(* Logix 5000 Rung export; software revision 16.04 *)

MODULES
   Local : vendor None type None code None
   MVI69E_AFC : vendor None type None code None
END_MODULES

TYPE AFCESiteAlarms :   // Indicates if a meter has any alarms
STRUCT
   Meter1 : BOOL;   // Meter in alarm
   Meter2 : BOOL;   // Meter in alarm
   Meter3 : BOOL;   // Meter in alarm
   Meter4 : BOOL;   // Meter in alarm
   Meter5 : BOOL;   // Meter in alarm
   Meter6 : BOOL;   // Meter in alarm
   Meter7 : BOOL;   // Meter in alarm
   Meter8 : BOOL;   // Meter in alarm
   Meter9 : BOOL;   // Meter in alarm
   Meter10 : BOOL;   // Meter in alarm
   Meter11 : BOOL;   // Meter in alarm
   Meter12 : BOOL;   // Meter in alarm
   Meter13 : BOOL;   // Meter in alarm
   Meter14 : BOOL;   // Meter in alarm
   Meter15 : BOOL;   // Meter in alarm
   Meter16 : BOOL;   // Meter in alarm
END_STRUCT
END_TYPE

TYPE AFCEFlag :   // Flags contains status information updated by ladder and also trigger bits for clock update
STRUCT
   AFCStopped : BOOL;   // Indicates that the module has sent a new input block to be processed by ladder - UPDATED BY LADDER
   AFCInputSequenceNum : INT;   // Meter number (0 -15) associated to blocks 1-16. Used to update "Profile" (meter type and product group.) UPDATED BY LADDER
END_STRUCT
END_TYPE

TYPE AFCEUtilBlockNonInterrupt :
STRUCT
   Now : BOOL;
   ModbusMasterCommand : BOOL;
   ModbusMasterResponse : BOOL;
   Archive : DINT;
   Prover : BOOL;
   PassThru : BOOL;
   Calibration : BOOL;
END_STRUCT
END_TYPE

TYPE AFCEProveConfigEnable :   // Prove controls at enable
STRUCT
   MeterNumber : INT;   // Meter number requested (1-16)
   AutoAcceptProve : BOOL;   // Auto-accept the prove
   AutoContinueProve : BOOL;   // Auto-continue the prove
END_STRUCT
END_TYPE

TYPE AFCEModbusGateway :   // Modbus Gateway
STRUCT
   Command : AFCEModbusGatewayCommand[10];   // Modbus gateway commands - contains setup and modbus data
END_STRUCT
END_TYPE

TYPE AFCEModbusMasterDataType :   // Modbus master data type
STRUCT
   Bit : BOOL;   // bit type
   Word : BOOL;   // word type (16-bit)
   Long : BOOL;   // long integer (32-bit)
   LongRemote : BOOL;   // long integer (32-bit)
END_STRUCT
END_TYPE

TYPE AFCEUtil :   // Used for internal ladder logic usage. These values must not be changed by user application.
STRUCT
   Flags : AFCEFlag;   // Wallclock update commands
   CycleCounter : INT;   // Reflects current block ID calculated by ladder to be sent to the module
   Buffer : AFCEUtilBuffer;
   Block : AFCEUtilBlock;
END_STRUCT
END_TYPE

TYPE AFCEWallclock :
STRUCT
   GetAFCTime : BOOL;   // Get current AFC Time
   SetAFCTimeFromPLCTime : BOOL;   // Set AFC time from PLC time. Updates current AFC time
   EnableLocalDateTime : BOOL;   // Enable Local Date Time.
   AFCTime : AFCETime;   // Coordinated Universal Time. Updated by either getting or setting AFC time.
END_STRUCT
END_TYPE

TYPE AFCEProvePhaseBitmap :   // AFC prove phase bitmap
STRUCT
   NotSelected : BOOL;   // Not selected
   Active : BOOL;   // Active, not counting
   CountingPast1stSwitch : BOOL;   // Counting past 1st switch for Udir and forward leg for Bdir)
   Past2ndSwitchFwdLeg : BOOL;   // Past 2nd switch forward leg (bidirectional only)
   Past1stSwithRetLeg : BOOL;   // Past 1st switch return leg (bidirectional only)
   RunComplete : BOOL;   // Run complete. past 2nd switch.
END_STRUCT
END_TYPE

TYPE AFCEProveInputConfig :   // Prove input block results - prover configuration
STRUCT
   Type : INT;   // Prover type
   Options : INT;   // Prover options
   RunsPerProveTotal : INT;   // Total runs per prove
   RunsPerProveSelected : INT;   // Selected runs per prove
   MaxRunsBeforeAbort : INT;   // Max total runs before abort
   ShortPassesPerRun : INT;   // Short passes per run if bidir = 2 , else 0
END_STRUCT
END_TYPE

TYPE AFCEModbusGatewayCommand :   // Modbus Gateway Command
STRUCT
   Config : AFCEModbusGatewayConfig;   // Config data to be entered by the user.
   Trigger : BOOL;   // Trigger the Command, when cleared module has responded.
   Data : INT[200];   // Contains modbus data written to the module (write commands)
END_STRUCT
END_TYPE

TYPE AFCEProveConfigAccept :   // Prove controls at accept. If auto-accept is selected must be available at enable
STRUCT
   RequestedInterpolationPoint : INT;   // Requested interpolation point (0 nearest)
   ApplyMFChangeAllStreams : BOOL;   // Apply change in meter factor to all streams
   ApplyMFChangeCurve : BOOL;   // Apply change in meter factor to all curve points
   ApplyNewMF : BOOL;   // CApply new meter factor
END_STRUCT
END_TYPE

TYPE AFCEModbusMasterCommand :   // Modbus Master Command
STRUCT
   Config : AFCEModbusMasterConfig;   // Modbus Master Configuration
   ErrorCode : INT;   // Error Code associated to Modbus Master Command
   Pending : BOOL;   // Pending Modbus Master Command - waiting for Modbus Response
   ReturnedTransactionID : DINT;   // Changes to Config.TransactionID value when response has returned.
   Data : INT[100];   // Read or Write Data
END_STRUCT
END_TYPE

TYPE AFCEProveSequencing :   // AFC prove sequencing tag for phase selection and ball positioning
STRUCT
   Phase : AFCEProvePhaseBitmap;   // AFC phase sequencing
   BallPositionReady : BOOL;   // Ball position: Ready (Udir & Bdir only; fwd leg Bdir)
   BallPositionSealed : BOOL;   // Ball position: Sealed (Udir & Bdir only; fwd leg Bdir)
   BallPositionReadyBwdLeg : BOOL;   // Ball position: Ready bwd leg (Bdir only)
   BallPositionSealedBwdLeg : BOOL;   // Ball position: Sealed bwd leg (Bdir only)
END_STRUCT
END_TYPE

TYPE AFCEUtilBlockInterrupt :
STRUCT
   Now : BOOL;
   ModbusGateway : DINT;
   EnableDisable : BOOL;
   Analysis : DINT;
END_STRUCT
END_TYPE

TYPE AFCEUtilBlock :
STRUCT
   ProcessInput : INT;
   InterruptPending : AFCEUtilBlockInterrupt;
   InterruptComplete : AFCEUtilBlockInterrupt;
   NonInterruptPending : AFCEUtilBlockNonInterrupt;
   NonInterruptComplete : AFCEUtilBlockNonInterrupt;
END_STRUCT
END_TYPE

TYPE AFCEModbusGatewayConfig :   // Modbus Ggateway Configuration
STRUCT
   Enable : BOOL;   // Set to 1 to enable modbus gateway command (0=disable)
   StartRegister : DINT;   // Start modbus address
   RegisterCount : INT;   // Word count (200 max)
   FunctionType : BOOL;   // 0 = read command, 1 = write command
   RegisterType : BOOL;   // 0 = holding register, 1 = input register
   SlaveType : BOOL;   // 0 = primary slave, 1 = virtual slave
END_STRUCT
END_TYPE

TYPE AFCEModbusPassThru :   // AFC Modbus Pass-thru
STRUCT
   Enable : BOOL;   // Set to 1 to enable pass-thru functionality (requires AFC Manager setting)
   MessagePresent : BOOL;   // Message present in the response block
   GetMessage : BOOL;   // Get the pass-thru message. When the bit is cleared the message has been transferred to the PLC.
   FunctionBitWrite : BOOL;   // Function bit write
   OverflowError : BOOL;   // Overflow error flag
   ModbusAddress : INT;   // Destination modbus address
   RegisterCount : INT;   // Number of elements associated to command
   ReadDataWord : INT[125];   // Contains received data for word commands
   ReadDataBit : AFCEModbusPassThruBitData;   // Contains received data for bit commands
END_STRUCT
END_TYPE

TYPE AFCEUtilBuffer :   // Buffer
STRUCT
   Input : INT[248];   // Input buffer contains the complete block to be copied from the module
   Output : INT[247];   // Output buffer contains data the complete block to be copied to the module
   Process : INT[180];
   ArchiveDay : INT[98];
   ArchiveHour : INT[98];
   Prove : INT[26];
   Analysis : INT[198];
   MeterEnableDisable : INT[4];
   StreamEnable : INT[36];
   StreamDisable : INT[36];
   StreamSelect : INT[24];
   MeterSignals : INT[24];
   Calibration : INT[36];
END_STRUCT
END_TYPE

TYPE AFCEProveStatus :   // Status of the prove (returned from the module to the processor)
STRUCT
   ProveAccepted : BOOL;   // Prove was accepted
   MeterFactorApplied : BOOL;   // Meter factor was applied
   MFAppliedToCurve : BOOL;   // Meter factor was applied to all points in the curve
   MFAppliedToStreams : BOOL;   // Meter factor was applied to all streams
   ProveRejectedByCommand : BOOL;   // Prove was rejected by command
   ProveRejectedNoRuns : BOOL;   // Prove was rejected - empty prove (no runs)
   ProveRejectedDivideBy0 : BOOL;   // Prove was rejected - divide by 0
   ProveEnabled : BOOL;   // Prove is enabled
   ProvingRunInProgress : BOOL;   // Proving run is in progress
   ProveRejectedAbort : BOOL;   // Prove rejected: abort
   ProvePaused : BOOL;   // Prove is paused
   RunCancelled : BOOL;   // Run Is cancelled
   RunTimedOut : BOOL;   // Run timed out
END_STRUCT
END_TYPE

TYPE AFCEProveConfig :   // Controls (configuration settings) associated to the prover
STRUCT
   Enable : AFCEProveConfigEnable;   // Controls at enable
   Accept : AFCEProveConfigAccept;   // Controls at accept
END_STRUCT
END_TYPE

TYPE AFCESiteStatus :   // Site status bits - contains general information about the module - not meter specific
STRUCT
   AFCActive : BOOL;   // AFC active
   ChecksumAlarms : BOOL;   // Checkum alarm active
   Reserved2 : BOOL;
   Reserved3 : BOOL;
   PLCHalted : BOOL;   // PLC in program mode or missing
   CfgChanged : BOOL;   // Configuration changed
   Powerup : BOOL;   // Module powered up
   ColdStart : BOOL;   // Module performed cold start (BBRAM initialized)
   ModbusMasterPending : BOOL;   // Modbus Master Poll Pending
   ModbusMasterComplete : BOOL;   // Modbus Master Poll Complete
   ModbusPassThruPending : BOOL;   // Modbus Pass-thru Input Pending
   CalibrationRequest : BOOL;   // Calibration request from module
   ProverEnabled : BOOL;   // Prover Enabled
   Reserved13 : BOOL;
   Reserved14 : BOOL;
   Reserved15 : BOOL;
END_STRUCT
END_TYPE

TYPE AFCEModbusMaster :   // Modbus Master. Port 3 must be configured as modbus master through AFC Manager to use this feature.
STRUCT
   Enable : BOOL;   // Enable the modbus master funcionality
   CommandIndex : INT;   // Selects which command index will be executed
   Command : AFCEModbusMasterCommand[10];   // Each command contains a specific modbus request to be sent out of the port
END_STRUCT
END_TYPE

TYPE AFCEProveProcess :   // Prove process output from processor to the module
STRUCT
   Sequencing : AFCEProveSequencing;   // Prover sequencing
   Temperature : REAL;   // Temperature for Single Probe provers. And Inlet Temperature for Dual Probe Provers.
   OutletTemperature : REAL;   // Outlet Temperature for Provers with Dual Probes.
   SwitchBarTemperature : REAL;   // Switch bar temperature
   Pressure : REAL;   // Pressure for Single Probe provers. And Inlet Pressure for Dual Probe Provers.
   OutletPressure : REAL;   // Outlet Pressure for Provers with Dual Probes.
   ProverDensity : REAL;   // Prover density
END_STRUCT
END_TYPE

TYPE AFCETime :   // AFC time format used for wallclock update.
STRUCT
   Year : DINT;   // Year
   Month : DINT;   // Month
   Day : DINT;   // Day
   Hour : DINT;   // Hour
   Minute : DINT;   // Minute
   second : DINT;   // Seconds
END_STRUCT
END_TYPE

TYPE AFCEModbusMasterSwap :   // Modbus master swap words/ swap bytes
STRUCT
   SwapWords : BOOL;   // Swap words
   SwapBytes : BOOL;   // Swap bytes
END_STRUCT
END_TYPE

TYPE AFCEProvePulseCount :   // Values to be supplied at the end of the pass/run
STRUCT
   Meter : DINT;   // Meter pulse count
   MasterMeter : DINT;   // Master meter pulse count
END_STRUCT
END_TYPE

TYPE AFCEModbusPassThruBitData :   // AFC Modbus Pass-thru Bit Data
STRUCT
   Data : BOOL[2016];   // Contains received data for bit commands
END_STRUCT
END_TYPE

TYPE AFCEModbusMasterConfig :   // Modbus master command settings
STRUCT
   Enable : BOOL;   // Set to 1 to enable command (0=disable)
   FunctionType : BOOL;   // Set to 1 to select write command (0=read command)
   RegisterBank : BOOL;   // Set to 1 to select input register (0=holding register)
   DataType : AFCEModbusMasterDataType;   // Select data type format
   SwapOption : AFCEModbusMasterSwap;   // Select byte and word swap (1 = swap, 0 = no swap)
   TypeSwap : INT;   // This value is calculated by ladder logic and must not be modified by user
   SlaveAddress : INT;   // Modbus slave address of remote device
   ModbusAddress : INT;   // Modbus data address on remote slave
   ElementCount : INT;   // Number of data elements (125 words)
   TransactionID : INT;   // Transaction ID. This value is returned to the ReturnedTransaction ID when the response has been received.
END_STRUCT
END_TYPE

TYPE AFCEModuleDef :   // Main user defined data type
STRUCT
   ModbusGateway : AFCEModbusGateway;   // Reads and write data between processor and module modbus table
   ModbusMaster : AFCEModbusMaster;   // Setup modbus master commands to be sent to remote slaves (through Port 3)
   ModbusPassThru : AFCEModbusPassThru;   // Modbus pass-thru data
   SiteStatus : AFCESiteStatus;   // Site status
   MeterAlarms : AFCESiteAlarms;   // Meter Alarms
   Prove : AFCEProve;   // Prover
   Wallclock : AFCEWallclock;   // Set clock and get clock information
   Firmware : AFCEFirmwareVersion;   // Firmware information
   Util : AFCEUtil;   // Used by ladder logic
END_STRUCT
END_TYPE

TYPE AFCEProveSignals :   // Contains the proving signals that will trigger specific tasks from the module
STRUCT
   EnableProve : BOOL;   // Enables the prove
   AcceptProve : BOOL;   // Accepts the prove
   RejectProve : BOOL;   // Reject the prove
   RunStart : BOOL;   // Starts the run
   RunComplete : BOOL;   // Flags that the run is complete
   RunCancel : BOOL;   // Cancels the run
   RunDelete : BOOL;   // Deletes the run
   PassComplete : BOOL;   // Flag that the pass is complete
   PauseProve : BOOL;   // Pauses the Proving Process
   AbortProve : BOOL;   // Aborts the prove
END_STRUCT
END_TYPE

TYPE AFCEFirmwareVersion :
STRUCT
   Major : SINT;   // Major Version number
   Minor : SINT;   // Minor Version number
   Revision : INT;   // Revision
END_STRUCT
END_TYPE

TYPE AFCEProveRunResults :   // Run results of the prove. Copied from the module to the pocessor
STRUCT
   CountAttempted : INT;   // Run count attempted
   CountCompleted : INT;   // Run count completed
   CountSelected : INT;   // Run count selected
   RunsSelected : INT;   // Bit Mapped Runs selected for calculations from completed runs
   NewMeterFactor : REAL;   // New meter factor
   ChangeInMeterFactor : REAL;   // Change in meter factor
END_STRUCT
END_TYPE

TYPE AFCEProve :   // Prove
STRUCT
   Process : AFCEProveProcess;   // Process Variables
   Signals : AFCEProveSignals;   // AFC Prove Signals (triggers the proving update)
   Config : AFCEProveConfig;   // AFC Prove Control (configuration settings)
   PulseCounts : AFCEProvePulseCount;   // Pulse counts to be updated at the end of the run/pass
   ConfigInput : AFCEProveInputConfig;   // AFC prover input configuration
   Status : AFCEProveStatus;   // AFC prover status
   ErrorCode : INT;   // Prove error code
   ProveControlsEcho : INT;   // AFC module Echos the state of the Prove Controls
   RequestedMeterEcho : INT;   // AFC module Echos the Meter number requested
   RequestedCurvePointEcho : INT;   // AFC module Echos the requested Curve Point
   RunResults : AFCEProveRunResults;   // Prove and run results
   ProveEnabled : BOOL;   // ON if prove is enabled. This flag is coped from inputbuffer[247]
END_STRUCT
END_TYPE

ADD_ON_INSTRUCTION AOI69EAFC   (* revision 1.5, vendor ProSoft Technology Inc., ExecutePrescan *)
// Add-On instruction for the MVI69E-AFC.
// Module Interface.
// Revision note:
// Made changes to the ModbusGatewayConfig UDT StartRegister Tag Data Type from INT to DINT.
// Help:
// Compatible with version 4.04 of MVI69E-AFC firmware or higher.
// v1.3: Option to choose LocalDateTime.
// v1.4: Changed Prescan FLL instruction length from 240 words to 180 for proccess inputs. This stopped mismatch issue
// v1.4: Changed COP instruction length from 240 words to 180 on rung 19 for procces inputs to output block. Modified ProfileBlockID INT to DINT.
// v1.5: Made changes to the ModbusGatewayConfig UDT StartRegister Tag Data Type from INT to DINT.
VAR_IN_OUT
   ConnectionInput : INT[248]; {required}
   ConnectionOutput : INT[247]; {required}
   AFC : AFCEModuleDef; {required}
        .UTIL.BUFFER.PROVE[12]   // Main user defined data type Buffer
END_VAR
VAR
   WallclockCurrentPLCTime : DINT[7];
   UTCTimeDelta : DINT;
   TimeZoneString : STRING;
   StoppedTimer : TIMER;
   ProverSignals : DINT;
   ProverPhase : DINT;
   ProverControls : DINT;
   ProveEnabled : BOOL;
   ProfileBlockID : DINT;
   ModbusMasterOutput : INT;
   CycleCounterPreviousStopped : INT;
   Offset1 : DINT;
   NotStoppedTimer : TIMER;
   ModbusPassThruOverflowError : BOOL;
   ModbusPassThruOutput : DINT;
   ModbusPassThruMessagePresent : BOOL;
   ModbusPassThruFunctionBitWrite : BOOL;
   ModbusMasterTransactionNumber : DINT;
   ModbusMasterReadWrite : BOOL;   // 0=Read 1=Write
   ModbusMasterPending : BOOL;
   ModbusMasterLongCount : DINT;
   ModbusGatewayReadWrite : BOOL;   // 0=Read, 1=Write
   ModbusGatewayOutput : DINT;
   ModbusGatewayIndexBitPosition : DINT;
   ModbusGatewayIndex : DINT;
   MJFAULTS : DINT[12];
   LocalHourChange : DINT;
   LatchStopped : BOOL;
   ForceReset : BOOL;
   AvoidBufferOverflowFault : DINT;   // Need this to prevent Overflow Minor Fault
   AFCTime : AFCETime;
END_VAR

ROUTINE Logic   (* ladder *)
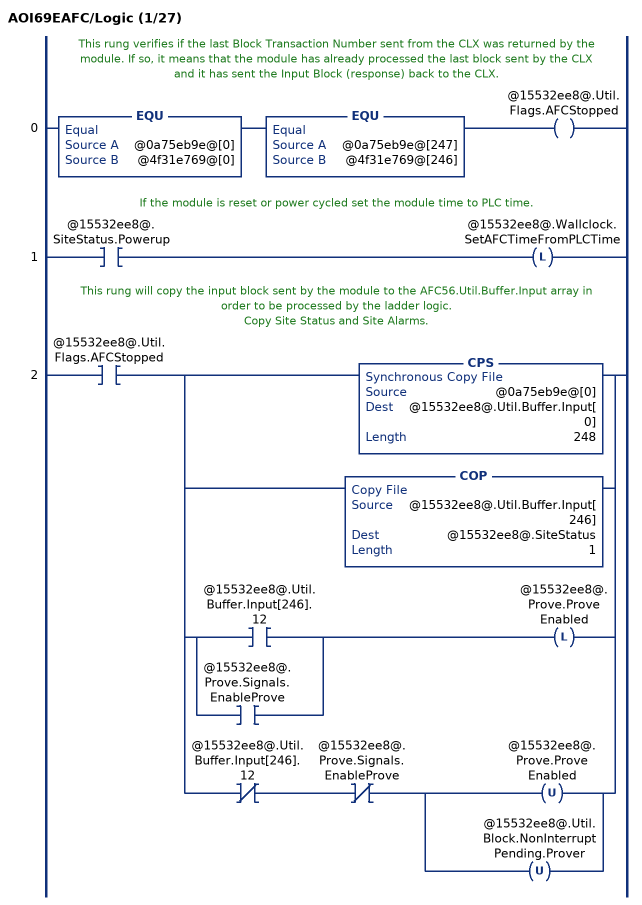
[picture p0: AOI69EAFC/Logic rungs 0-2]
   // This rung verifies if the last Block Transaction Number sent from the CLX was returned by the module. If so, it means that the module has already processed the last block sent by the CLX and it has sent the Input Block (response) back to the CLX.
   0: EQU(@0a75eb9e@[0],@4f31e769@[0])EQU(@0a75eb9e@[247],@4f31e769@[246])OTE(@15532ee8@.Util.Flags.AFCStopped);
   // If the module is reset or power cycled set the module time to PLC time.
   1: XIC(@15532ee8@.SiteStatus.Powerup)OTL(@15532ee8@.Wallclock.SetAFCTimeFromPLCTime);
   // This rung will copy the input block sent by the module to the AFC56.Util.Buffer.Input array in order to be processed by the ladder logic.
   // Copy Site Status and Site Alarms.
   2: XIC(@15532ee8@.Util.Flags.AFCStopped)[CPS(@0a75eb9e@[0],@15532ee8@.Util.Buffer.Input[0],248) ,COP(@15532ee8@.Util.Buffer.Input[246],@15532ee8@.SiteStatus,1) ,[XIC(@15532ee8@.Util.Buffer.Input[246].12) ,XIC(@15532ee8@.Prove.Signals.EnableProve) ] OTL(@15532ee8@.Prove.ProveEnabled) ,XIO(@15532ee8@.Util.Buffer.Input[246].12) XIO(@15532ee8@.Prove.Signals.EnableProve) [OTU(@15532ee8@.Prove.ProveEnabled) ,OTU(@15532ee8@.Util.Block.NonInterruptPending.Prover) ] ];
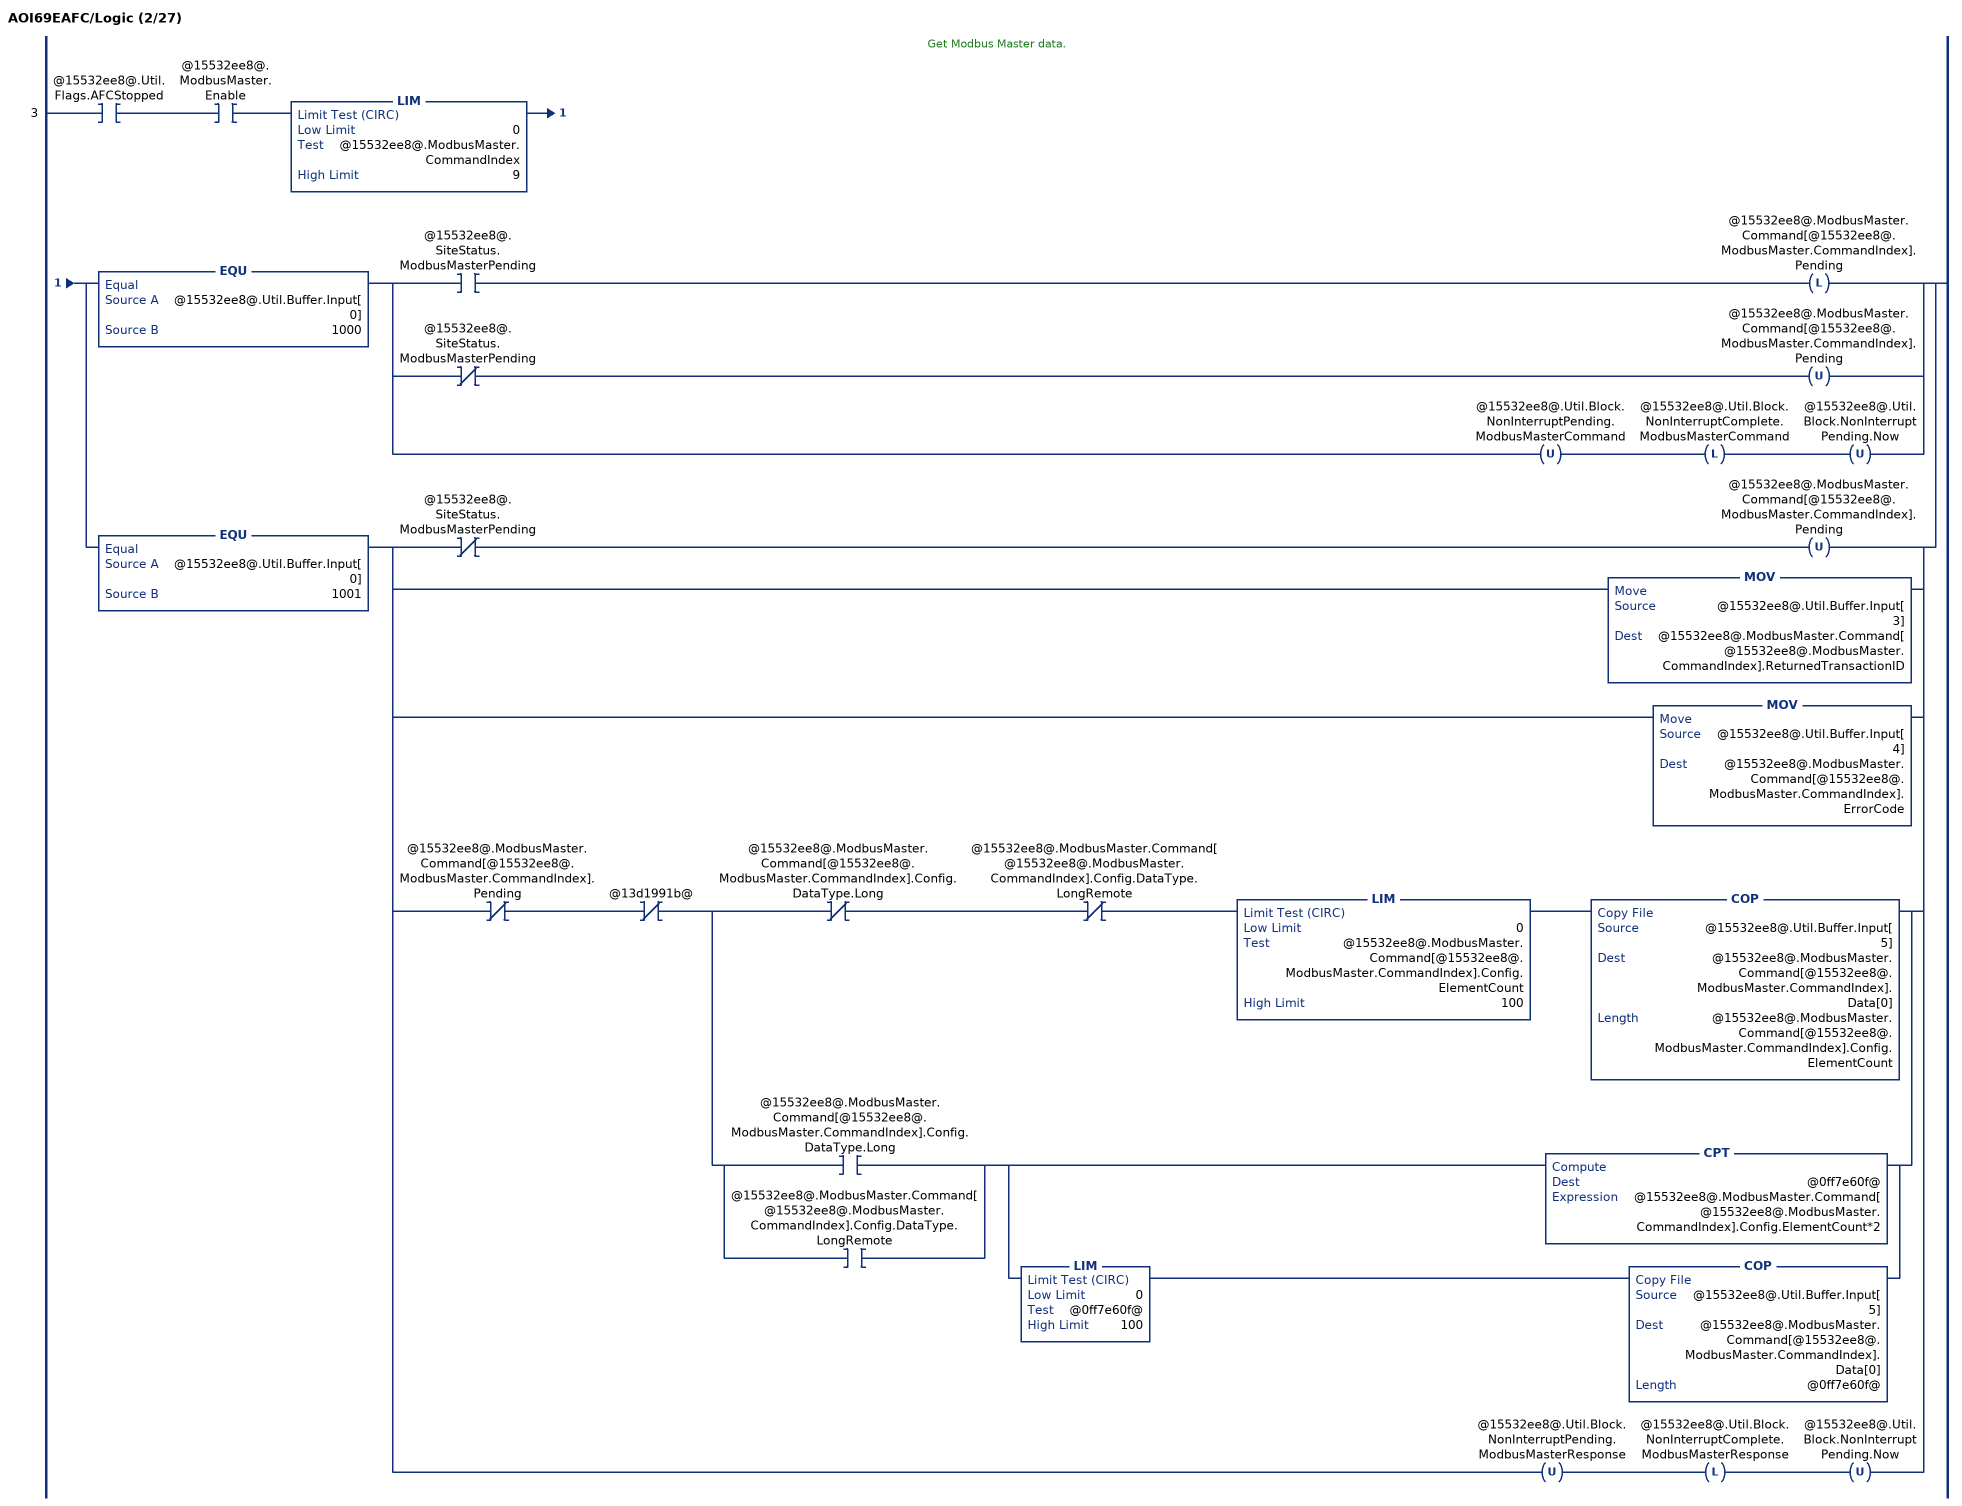
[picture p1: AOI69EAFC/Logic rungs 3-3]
   // Get Modbus Master data.
   3: XIC(@15532ee8@.Util.Flags.AFCStopped)XIC(@15532ee8@.ModbusMaster.Enable)LIM(0,@15532ee8@.ModbusMaster.CommandIndex,9)[EQU(@15532ee8@.Util.Buffer.Input[0],1000) [XIC(@15532ee8@.SiteStatus.ModbusMasterPending) OTL(@15532ee8@.ModbusMaster.Command[@15532ee8@.ModbusMaster.CommandIndex].Pending) ,XIO(@15532ee8@.SiteStatus.ModbusMasterPending) OTU(@15532ee8@.ModbusMaster.Command[@15532ee8@.ModbusMaster.CommandIndex].Pending) ,OTU(@15532ee8@.Util.Block.NonInterruptPending.ModbusMasterCommand) OTL(@15532ee8@.Util.Block.NonInterruptComplete.ModbusMasterCommand) OTU(@15532ee8@.Util.Block.NonInterruptPending.Now) ] ,EQU(@15532ee8@.Util.Buffer.Input[0],1001) [XIO(@15532ee8@.SiteStatus.ModbusMasterPending) OTU(@15532ee8@.ModbusMaster.Command[@15532ee8@.ModbusMaster.CommandIndex].Pending) ,MOV(@15532ee8@.Util.Buffer.Input[3],@15532ee8@.ModbusMaster.Command[@15532ee8@.ModbusMaster.CommandIndex].ReturnedTransactionID) ,MOV(@15532ee8@.Util.Buffer.Input[4],@15532ee8@.ModbusMaster.Command[@15532ee8@.ModbusMaster.CommandIndex].ErrorCode) ,XIO(@15532ee8@.ModbusMaster.Command[@15532ee8@.ModbusMaster.CommandIndex].Pending) XIO(@13d1991b@) [XIO(@15532ee8@.ModbusMaster.Command[@15532ee8@.ModbusMaster.CommandIndex].Config.DataType.Long) XIO(@15532ee8@.ModbusMaster.Command[@15532ee8@.ModbusMaster.CommandIndex].Config.DataType.LongRemote) LIM(0,@15532ee8@.ModbusMaster.Command[@15532ee8@.ModbusMaster.CommandIndex].Config.ElementCount,100) COP(@15532ee8@.Util.Buffer.Input[5],@15532ee8@.ModbusMaster.Command[@15532ee8@.ModbusMaster.CommandIndex].Data[0],@15532ee8@.ModbusMaster.Command[@15532ee8@.ModbusMaster.CommandIndex].Config.ElementCount) ,[XIC(@15532ee8@.ModbusMaster.Command[@15532ee8@.ModbusMaster.CommandIndex].Config.DataType.Long) ,XIC(@15532ee8@.ModbusMaster.Command[@15532ee8@.ModbusMaster.CommandIndex].Config.DataType.LongRemote) ] [CPT(@0ff7e60f@,@15532ee8@.ModbusMaster.Command[@15532ee8@.ModbusMaster.CommandIndex].Config.ElementCount*2) ,LIM(0,@0ff7e60f@,100) COP(@15532ee8@.Util.Buffer.Input[5],@15532ee8@.ModbusMaster.Command[@15532ee8@.ModbusMaster.CommandIndex].Data[0],@0ff7e60f@) ] ] ,OTU(@15532ee8@.Util.Block.NonInterruptPending.ModbusMasterResponse) OTL(@15532ee8@.Util.Block.NonInterruptComplete.ModbusMasterResponse) OTU(@15532ee8@.Util.Block.NonInterruptPending.Now) ] ];
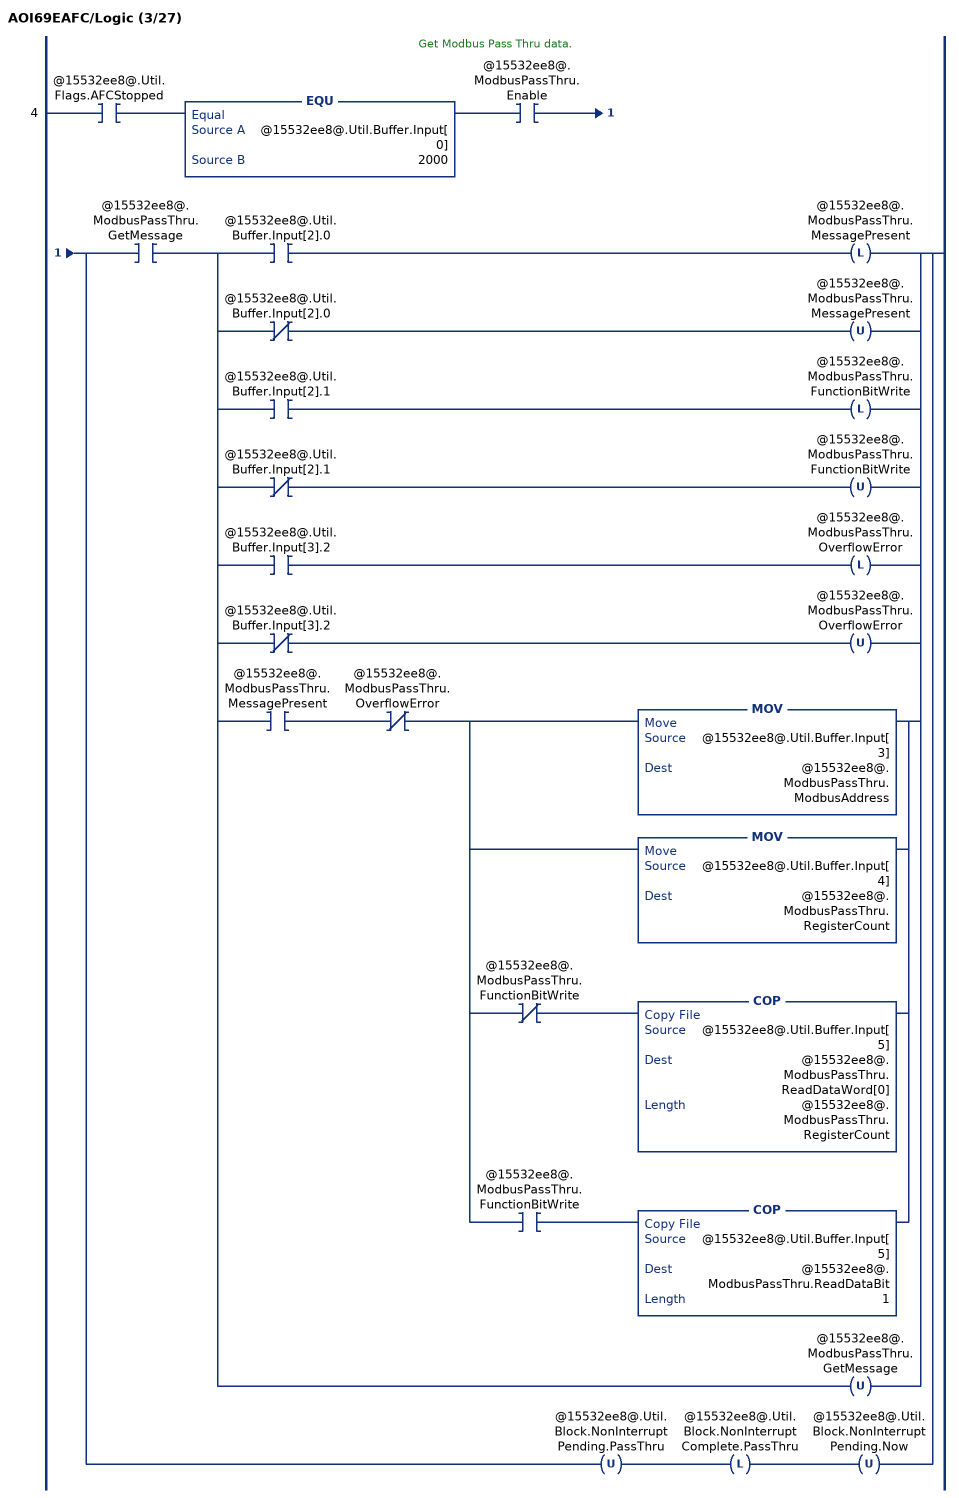
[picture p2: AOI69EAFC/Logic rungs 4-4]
   // Get Modbus Pass Thru data.
   4: XIC(@15532ee8@.Util.Flags.AFCStopped)EQU(@15532ee8@.Util.Buffer.Input[0],2000)XIC(@15532ee8@.ModbusPassThru.Enable)[XIC(@15532ee8@.ModbusPassThru.GetMessage) [[XIC(@15532ee8@.Util.Buffer.Input[2].0) OTL(@15532ee8@.ModbusPassThru.MessagePresent) ,XIO(@15532ee8@.Util.Buffer.Input[2].0) OTU(@15532ee8@.ModbusPassThru.MessagePresent) ,XIC(@15532ee8@.Util.Buffer.Input[2].1) OTL(@15532ee8@.ModbusPassThru.FunctionBitWrite) ,XIO(@15532ee8@.Util.Buffer.Input[2].1) OTU(@15532ee8@.ModbusPassThru.FunctionBitWrite) ,XIC(@15532ee8@.Util.Buffer.Input[3].2) OTL(@15532ee8@.ModbusPassThru.OverflowError) ,XIO(@15532ee8@.Util.Buffer.Input[3].2) OTU(@15532ee8@.ModbusPassThru.OverflowError) ] ,XIC(@15532ee8@.ModbusPassThru.MessagePresent) XIO(@15532ee8@.ModbusPassThru.OverflowError) [MOV(@15532ee8@.Util.Buffer.Input[3],@15532ee8@.ModbusPassThru.ModbusAddress) ,MOV(@15532ee8@.Util.Buffer.Input[4],@15532ee8@.ModbusPassThru.RegisterCount) ,XIO(@15532ee8@.ModbusPassThru.FunctionBitWrite) COP(@15532ee8@.Util.Buffer.Input[5],@15532ee8@.ModbusPassThru.ReadDataWord[0],@15532ee8@.ModbusPassThru.RegisterCount) ,XIC(@15532ee8@.ModbusPassThru.FunctionBitWrite) COP(@15532ee8@.Util.Buffer.Input[5],@15532ee8@.ModbusPassThru.ReadDataBit,1) ] ,OTU(@15532ee8@.ModbusPassThru.GetMessage) ] ,OTU(@15532ee8@.Util.Block.NonInterruptPending.PassThru) OTL(@15532ee8@.Util.Block.NonInterruptComplete.PassThru) OTU(@15532ee8@.Util.Block.NonInterruptPending.Now) ];
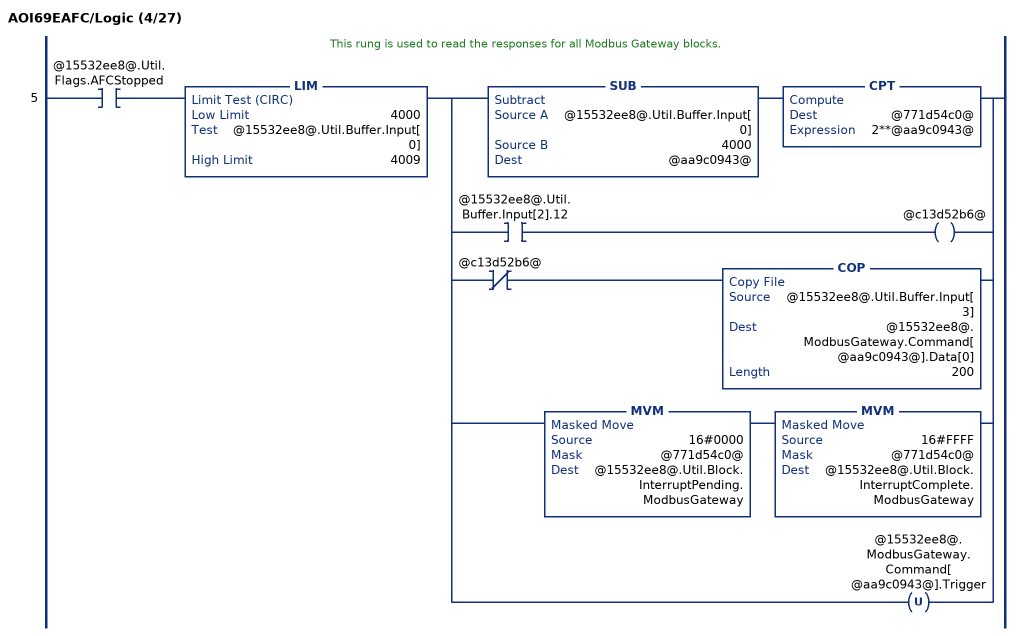
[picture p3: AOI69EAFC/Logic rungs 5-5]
   // This rung is used to read the responses for all Modbus Gateway blocks.
   5: XIC(@15532ee8@.Util.Flags.AFCStopped)LIM(4000,@15532ee8@.Util.Buffer.Input[0],4009)[SUB(@15532ee8@.Util.Buffer.Input[0],4000,@aa9c0943@) CPT(@771d54c0@,2**@aa9c0943@) ,XIC(@15532ee8@.Util.Buffer.Input[2].12) OTE(@c13d52b6@) ,XIO(@c13d52b6@) COP(@15532ee8@.Util.Buffer.Input[3],@15532ee8@.ModbusGateway.Command[@aa9c0943@].Data[0],200) ,MVM(16#0000,@771d54c0@,@15532ee8@.Util.Block.InterruptPending.ModbusGateway) MVM(16#FFFF,@771d54c0@,@15532ee8@.Util.Block.InterruptComplete.ModbusGateway) ,OTU(@15532ee8@.ModbusGateway.Command[@aa9c0943@].Trigger) ];
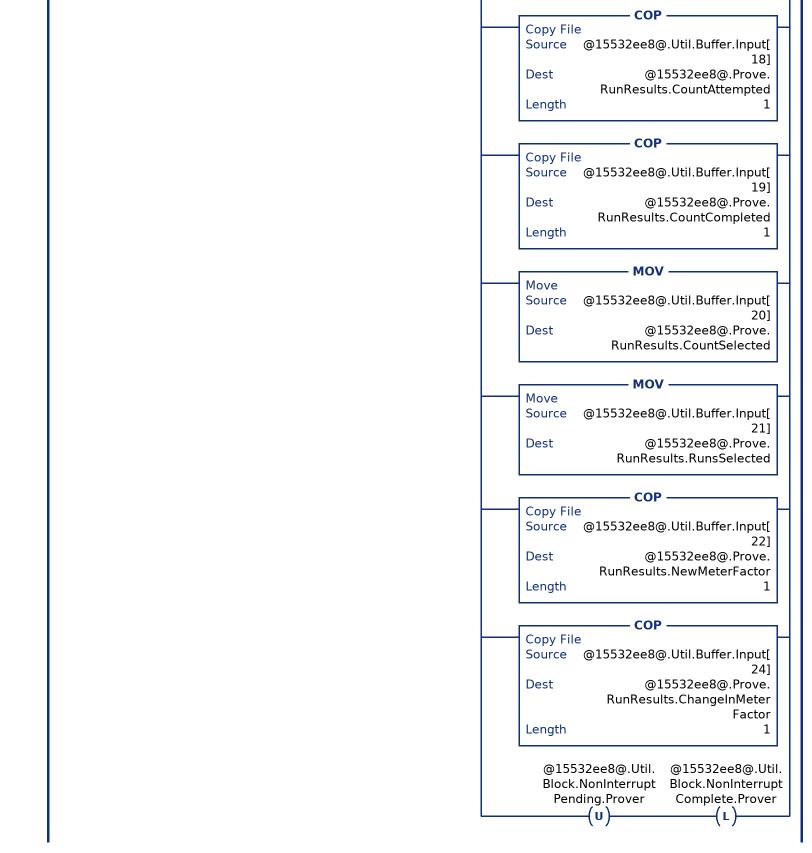
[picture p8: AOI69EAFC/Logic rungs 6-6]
   6: XIC(@15532ee8@.Util.Flags.AFCStopped)EQU(@15532ee8@.Util.Buffer.Input[0],5000)[XIC(@f8aaafbf@.1) OTU(@15532ee8@.Prove.Signals.EnableProve) ,XIC(@f8aaafbf@.2) OTU(@15532ee8@.Prove.Signals.AcceptProve) ,XIC(@f8aaafbf@.3) OTU(@15532ee8@.Prove.Signals.RejectProve) ,XIC(@f8aaafbf@.4) OTU(@15532ee8@.Prove.Signals.RunStart) ,XIC(@f8aaafbf@.5) OTU(@15532ee8@.Prove.Signals.RunComplete) ,XIC(@f8aaafbf@.6) OTU(@15532ee8@.Prove.Signals.RunCancel) ,XIC(@f8aaafbf@.7) OTU(@15532ee8@.Prove.Signals.RunDelete) ,XIC(@f8aaafbf@.9) OTU(@15532ee8@.Prove.Signals.PassComplete) ,XIC(@f8aaafbf@.12) OTU(@15532ee8@.Prove.Signals.PauseProve) ,XIC(@f8aaafbf@.14) OTU(@15532ee8@.Prove.Signals.AbortProve) ,MOV(@15532ee8@.Util.Buffer.Input[3],@15532ee8@.Prove.ConfigInput.Type) ,MOV(@15532ee8@.Util.Buffer.Input[4],@15532ee8@.Prove.ConfigInput.Options) ,MOV(@15532ee8@.Util.Buffer.Input[5],@15532ee8@.Prove.ConfigInput.RunsPerProveTotal) ,MOV(@15532ee8@.Util.Buffer.Input[6],@15532ee8@.Prove.ConfigInput.RunsPerProveSelected) ,MOV(@15532ee8@.Util.Buffer.Input[7],@15532ee8@.Prove.ConfigInput.MaxRunsBeforeAbort) ,MOV(@15532ee8@.Util.Buffer.Input[8],@15532ee8@.Prove.ConfigInput.ShortPassesPerRun) ,XIC(@15532ee8@.Util.Buffer.Input[12].0) OTL(@15532ee8@.Prove.Status.ProveAccepted) ,XIO(@15532ee8@.Util.Buffer.Input[12].0) OTU(@15532ee8@.Prove.Status.ProveAccepted) ,XIC(@15532ee8@.Util.Buffer.Input[12].1) OTL(@15532ee8@.Prove.Status.MeterFactorApplied) ,XIO(@15532ee8@.Util.Buffer.Input[12].1) OTU(@15532ee8@.Prove.Status.MeterFactorApplied) ,XIC(@15532ee8@.Util.Buffer.Input[12].2) OTL(@15532ee8@.Prove.Status.MFAppliedToCurve) ,XIO(@15532ee8@.Util.Buffer.Input[12].2) OTU(@15532ee8@.Prove.Status.MFAppliedToCurve) ,XIC(@15532ee8@.Util.Buffer.Input[12].3) OTL(@15532ee8@.Prove.Status.MFAppliedToStreams) ,XIO(@15532ee8@.Util.Buffer.Input[12].3) OTU(@15532ee8@.Prove.Status.MFAppliedToStreams) ,XIC(@15532ee8@.Util.Buffer.Input[12].4) OTL(@15532ee8@.Prove.Status.ProveRejectedByCommand) ,XIO(@15532ee8@.Util.Buffer.Input[12].4) OTU(@15532ee8@.Prove.Status.ProveRejectedByCommand) ,XIC(@15532ee8@.Util.Buffer.Input[12].5) OTL(@15532ee8@.Prove.Status.ProveRejectedNoRuns) ,XIO(@15532ee8@.Util.Buffer.Input[12].5) OTU(@15532ee8@.Prove.Status.ProveRejectedNoRuns) ,XIC(@15532ee8@.Util.Buffer.Input[12].6) OTL(@15532ee8@.Prove.Status.ProveRejectedDivideBy0) ,XIO(@15532ee8@.Util.Buffer.Input[12].6) OTU(@15532ee8@.Prove.Status.ProveRejectedDivideBy0) ,XIC(@15532ee8@.Util.Buffer.Input[12].8) OTL(@15532ee8@.Prove.Status.ProveEnabled) ,[XIO(@15532ee8@.Util.Buffer.Input[12].8) ,XIC(@f8aaafbf@.2) ,XIC(@f8aaafbf@.3) ,XIC(@f8aaafbf@.14) ] OTU(@15532ee8@.Prove.Status.ProveEnabled) ,XIC(@15532ee8@.Util.Buffer.Input[12].9) OTL(@15532ee8@.Prove.Status.ProvingRunInProgress) ,XIO(@15532ee8@.Util.Buffer.Input[12].9) OTU(@15532ee8@.Prove.Status.ProvingRunInProgress) ,XIC(@15532ee8@.Util.Buffer.Input[12].10) OTL(@15532ee8@.Prove.Status.ProvePaused) ,XIO(@15532ee8@.Util.Buffer.Input[12].10) OTU(@15532ee8@.Prove.Status.ProvePaused) ,XIC(@15532ee8@.Util.Buffer.Input[12].11) OTL(@15532ee8@.Prove.Status.RunCancelled) ,XIO(@15532ee8@.Util.Buffer.Input[12].11) OTU(@15532ee8@.Prove.Status.RunCancelled) ,XIC(@15532ee8@.Util.Buffer.Input[12].12) OTL(@15532ee8@.Prove.Status.RunTimedOut) ,XIO(@15532ee8@.Util.Buffer.Input[12].12) OTU(@15532ee8@.Prove.Status.RunTimedOut) ,XIC(@15532ee8@.Util.Buffer.Input[12].14) OTL(@15532ee8@.Prove.Status.ProveRejectedAbort) ,XIO(@15532ee8@.Util.Buffer.Input[12].14) OTU(@15532ee8@.Prove.Status.ProveRejectedAbort) ,MOV(@15532ee8@.Util.Buffer.Input[13],@15532ee8@.Prove.ErrorCode) ,MOV(@15532ee8@.Util.Buffer.Input[14],@15532ee8@.Prove.ProveControlsEcho) ,MOV(@15532ee8@.Util.Buffer.Input[15],@15532ee8@.Prove.RequestedMeterEcho) ,MOV(@15532ee8@.Util.Buffer.Input[17],@15532ee8@.Prove.RequestedCurvePointEcho) ,COP(@15532ee8@.Util.Buffer.Input[18],@15532ee8@.Prove.RunResults.CountAttempted,1) ,COP(@15532ee8@.Util.Buffer.Input[19],@15532ee8@.Prove.RunResults.CountCompleted,1) ,MOV(@15532ee8@.Util.Buffer.Input[20],@15532ee8@.Prove.RunResults.CountSelected) ,MOV(@15532ee8@.Util.Buffer.Input[21],@15532ee8@.Prove.RunResults.RunsSelected) ,COP(@15532ee8@.Util.Buffer.Input[22],@15532ee8@.Prove.RunResults.NewMeterFactor,1) ,COP(@15532ee8@.Util.Buffer.Input[24],@15532ee8@.Prove.RunResults.ChangeInMeterFactor,1) ,OTU(@15532ee8@.Util.Block.NonInterruptPending.Prover) OTL(@15532ee8@.Util.Block.NonInterruptComplete.Prover) ];
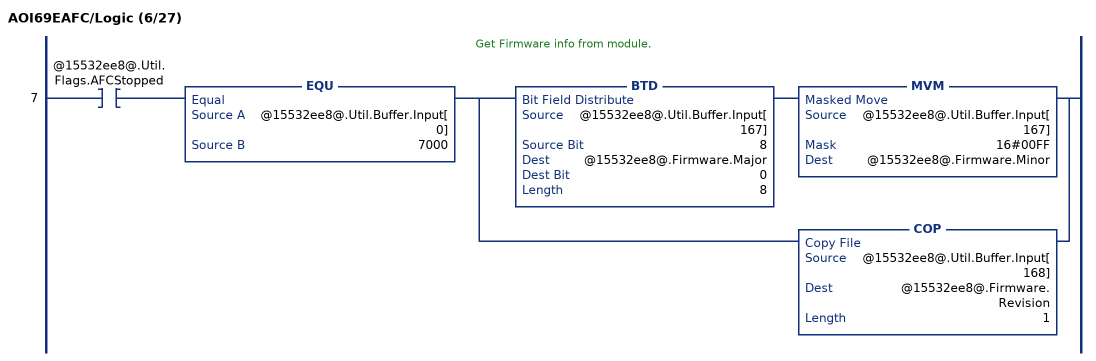
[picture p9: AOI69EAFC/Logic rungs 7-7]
   // Get Firmware info from module.
   7: XIC(@15532ee8@.Util.Flags.AFCStopped)EQU(@15532ee8@.Util.Buffer.Input[0],7000)[BTD(@15532ee8@.Util.Buffer.Input[167],8,@15532ee8@.Firmware.Major,0,8) MVM(@15532ee8@.Util.Buffer.Input[167],16#00FF,@15532ee8@.Firmware.Minor) ,COP(@15532ee8@.Util.Buffer.Input[168],@15532ee8@.Firmware.Revision,1) ];
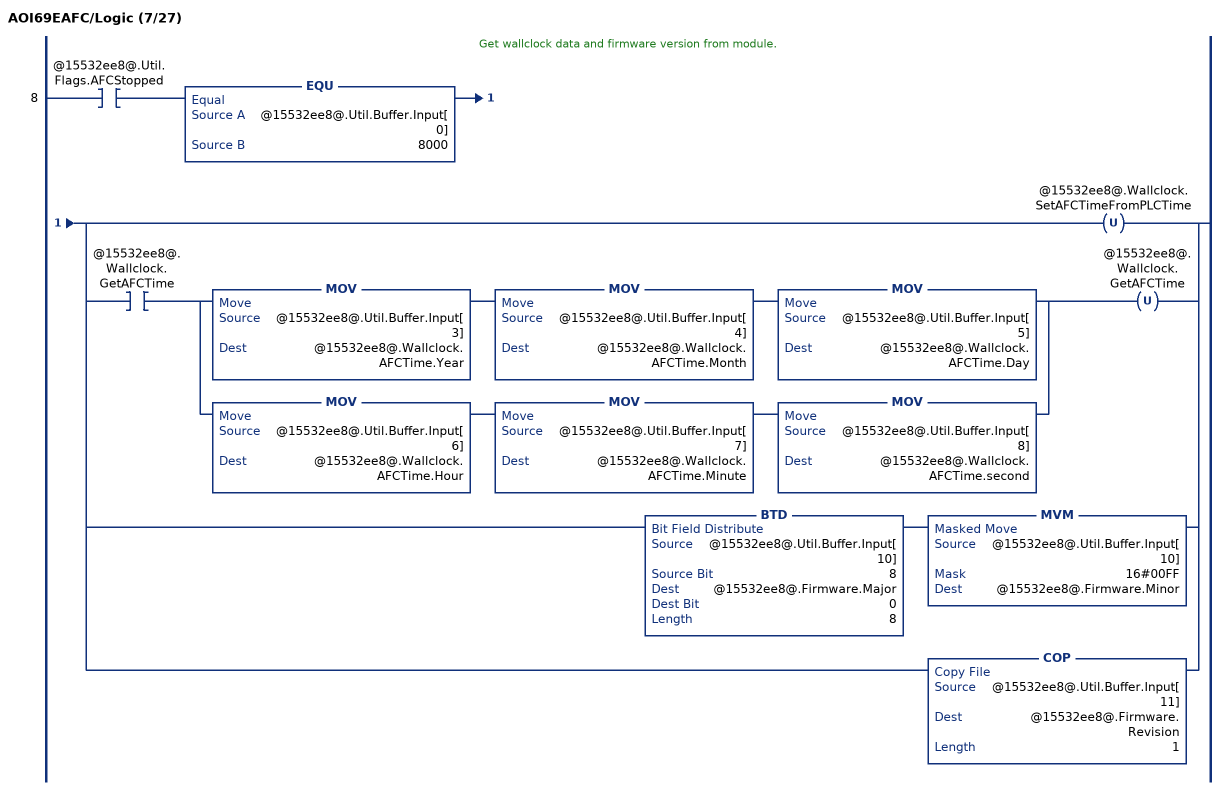
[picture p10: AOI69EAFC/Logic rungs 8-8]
   // Get wallclock data and firmware version from module.
   8: XIC(@15532ee8@.Util.Flags.AFCStopped)EQU(@15532ee8@.Util.Buffer.Input[0],8000)[OTU(@15532ee8@.Wallclock.SetAFCTimeFromPLCTime) ,XIC(@15532ee8@.Wallclock.GetAFCTime) [MOV(@15532ee8@.Util.Buffer.Input[3],@15532ee8@.Wallclock.AFCTime.Year) MOV(@15532ee8@.Util.Buffer.Input[4],@15532ee8@.Wallclock.AFCTime.Month) MOV(@15532ee8@.Util.Buffer.Input[5],@15532ee8@.Wallclock.AFCTime.Day) ,MOV(@15532ee8@.Util.Buffer.Input[6],@15532ee8@.Wallclock.AFCTime.Hour) MOV(@15532ee8@.Util.Buffer.Input[7],@15532ee8@.Wallclock.AFCTime.Minute) MOV(@15532ee8@.Util.Buffer.Input[8],@15532ee8@.Wallclock.AFCTime.second) ] OTU(@15532ee8@.Wallclock.GetAFCTime) ,[BTD(@15532ee8@.Util.Buffer.Input[10],8,@15532ee8@.Firmware.Major,0,8) MVM(@15532ee8@.Util.Buffer.Input[10],16#00FF,@15532ee8@.Firmware.Minor) ,COP(@15532ee8@.Util.Buffer.Input[11],@15532ee8@.Firmware.Revision,1) ] ];
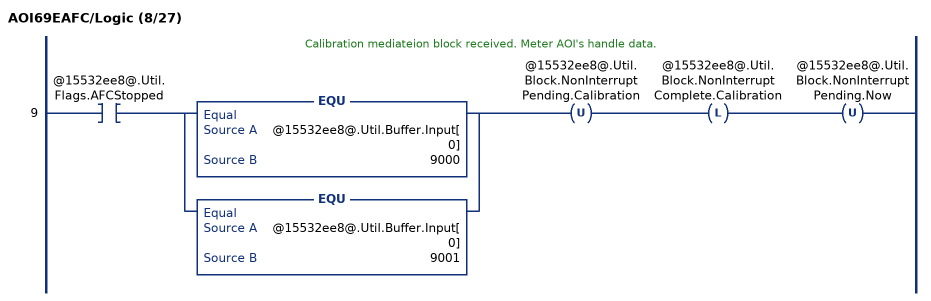
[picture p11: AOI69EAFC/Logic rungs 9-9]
   // Calibration mediateion block received. Meter AOI's handle data.
   9: XIC(@15532ee8@.Util.Flags.AFCStopped)[EQU(@15532ee8@.Util.Buffer.Input[0],9000) ,EQU(@15532ee8@.Util.Buffer.Input[0],9001) ]OTU(@15532ee8@.Util.Block.NonInterruptPending.Calibration)OTL(@15532ee8@.Util.Block.NonInterruptComplete.Calibration)OTU(@15532ee8@.Util.Block.NonInterruptPending.Now);
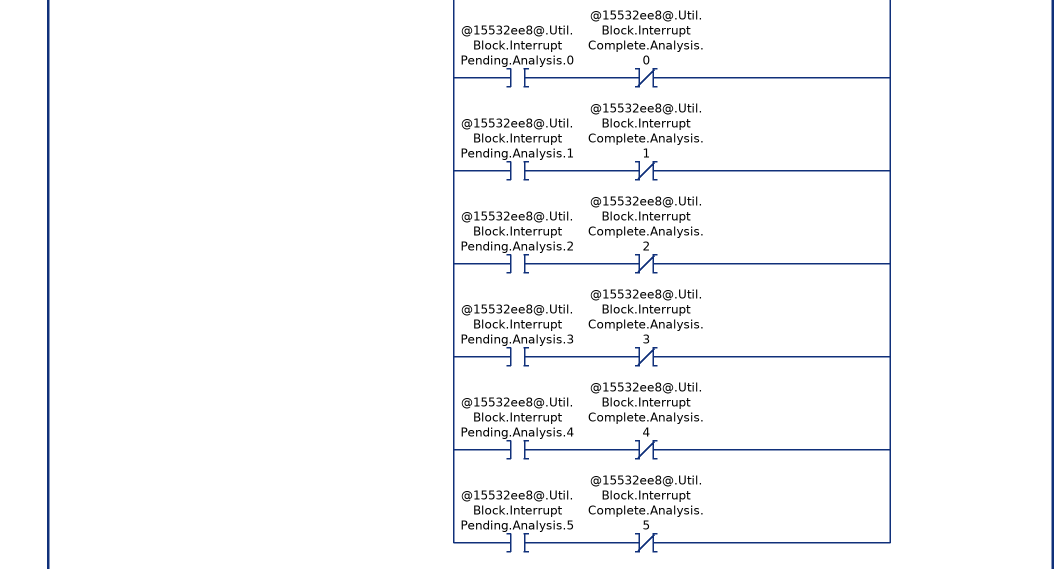
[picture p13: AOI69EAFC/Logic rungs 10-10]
   // Interrupt blocks (3000, 4000 and 7000) are interleaved between Process Input blocks.
   // Check if any interrupt block is pending.
   10: XIC(@15532ee8@.Util.Flags.AFCStopped)LIM(1,@15532ee8@.Util.Buffer.Input[0],11)[XIC(@15532ee8@.ModbusGateway.Command[0].Trigger) XIO(@15532ee8@.Util.Block.InterruptComplete.ModbusGateway.0) OTL(@15532ee8@.Util.Block.InterruptPending.ModbusGateway.0) ,XIC(@15532ee8@.ModbusGateway.Command[1].Trigger) XIO(@15532ee8@.Util.Block.InterruptComplete.ModbusGateway.1) OTL(@15532ee8@.Util.Block.InterruptPending.ModbusGateway.1) ,XIC(@15532ee8@.ModbusGateway.Command[2].Trigger) XIO(@15532ee8@.Util.Block.InterruptComplete.ModbusGateway.2) OTL(@15532ee8@.Util.Block.InterruptPending.ModbusGateway.2) ,XIC(@15532ee8@.ModbusGateway.Command[3].Trigger) XIO(@15532ee8@.Util.Block.InterruptComplete.ModbusGateway.3) OTL(@15532ee8@.Util.Block.InterruptPending.ModbusGateway.3) ,XIC(@15532ee8@.ModbusGateway.Command[4].Trigger) XIO(@15532ee8@.Util.Block.InterruptComplete.ModbusGateway.4) OTL(@15532ee8@.Util.Block.InterruptPending.ModbusGateway.4) ,XIC(@15532ee8@.ModbusGateway.Command[5].Trigger) XIO(@15532ee8@.Util.Block.InterruptComplete.ModbusGateway.5) OTL(@15532ee8@.Util.Block.InterruptPending.ModbusGateway.5) ,XIC(@15532ee8@.ModbusGateway.Command[6].Trigger) XIO(@15532ee8@.Util.Block.InterruptComplete.ModbusGateway.6) OTL(@15532ee8@.Util.Block.InterruptPending.ModbusGateway.6) ,XIC(@15532ee8@.ModbusGateway.Command[7].Trigger) XIO(@15532ee8@.Util.Block.InterruptComplete.ModbusGateway.7) OTL(@15532ee8@.Util.Block.InterruptPending.ModbusGateway.7) ,XIC(@15532ee8@.ModbusGateway.Command[8].Trigger) XIO(@15532ee8@.Util.Block.InterruptComplete.ModbusGateway.8) OTL(@15532ee8@.Util.Block.InterruptPending.ModbusGateway.8) ,XIC(@15532ee8@.ModbusGateway.Command[9].Trigger) XIO(@15532ee8@.Util.Block.InterruptComplete.ModbusGateway.9) OTL(@15532ee8@.Util.Block.InterruptPending.ModbusGateway.9) ,XIC(@15532ee8@.Util.Block.InterruptPending.EnableDisable) XIO(@15532ee8@.Util.Block.InterruptComplete.EnableDisable) ,XIC(@15532ee8@.Util.Block.InterruptPending.Analysis.0) XIO(@15532ee8@.Util.Block.InterruptComplete.Analysis.0) ,XIC(@15532ee8@.Util.Block.InterruptPending.Analysis.1) XIO(@15532ee8@.Util.Block.InterruptComplete.Analysis.1) ,XIC(@15532ee8@.Util.Block.InterruptPending.Analysis.2) XIO(@15532ee8@.Util.Block.InterruptComplete.Analysis.2) ,XIC(@15532ee8@.Util.Block.InterruptPending.Analysis.3) XIO(@15532ee8@.Util.Block.InterruptComplete.Analysis.3) ,XIC(@15532ee8@.Util.Block.InterruptPending.Analysis.4) XIO(@15532ee8@.Util.Block.InterruptComplete.Analysis.4) ,XIC(@15532ee8@.Util.Block.InterruptPending.Analysis.5) XIO(@15532ee8@.Util.Block.InterruptComplete.Analysis.5) ]OTL(@15532ee8@.Util.Block.InterruptPending.Now);
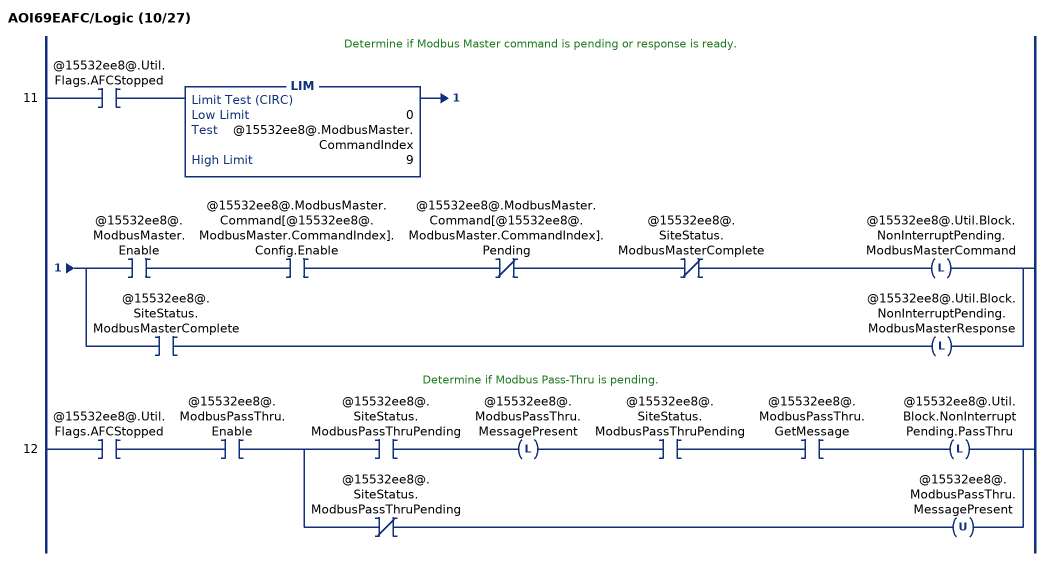
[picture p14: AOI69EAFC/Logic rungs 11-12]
   // Determine if Modbus Master command is pending or response is ready.
   11: XIC(@15532ee8@.Util.Flags.AFCStopped)LIM(0,@15532ee8@.ModbusMaster.CommandIndex,9)[XIC(@15532ee8@.ModbusMaster.Enable) XIC(@15532ee8@.ModbusMaster.Command[@15532ee8@.ModbusMaster.CommandIndex].Config.Enable) XIO(@15532ee8@.ModbusMaster.Command[@15532ee8@.ModbusMaster.CommandIndex].Pending) XIO(@15532ee8@.SiteStatus.ModbusMasterComplete) OTL(@15532ee8@.Util.Block.NonInterruptPending.ModbusMasterCommand) ,XIC(@15532ee8@.SiteStatus.ModbusMasterComplete) OTL(@15532ee8@.Util.Block.NonInterruptPending.ModbusMasterResponse) ];
   // Determine if Modbus Pass-Thru is pending.
   12: XIC(@15532ee8@.Util.Flags.AFCStopped)XIC(@15532ee8@.ModbusPassThru.Enable)[XIC(@15532ee8@.SiteStatus.ModbusPassThruPending) OTL(@15532ee8@.ModbusPassThru.MessagePresent) XIC(@15532ee8@.SiteStatus.ModbusPassThruPending) XIC(@15532ee8@.ModbusPassThru.GetMessage) OTL(@15532ee8@.Util.Block.NonInterruptPending.PassThru) ,XIO(@15532ee8@.SiteStatus.ModbusPassThruPending) OTU(@15532ee8@.ModbusPassThru.MessagePresent) ];
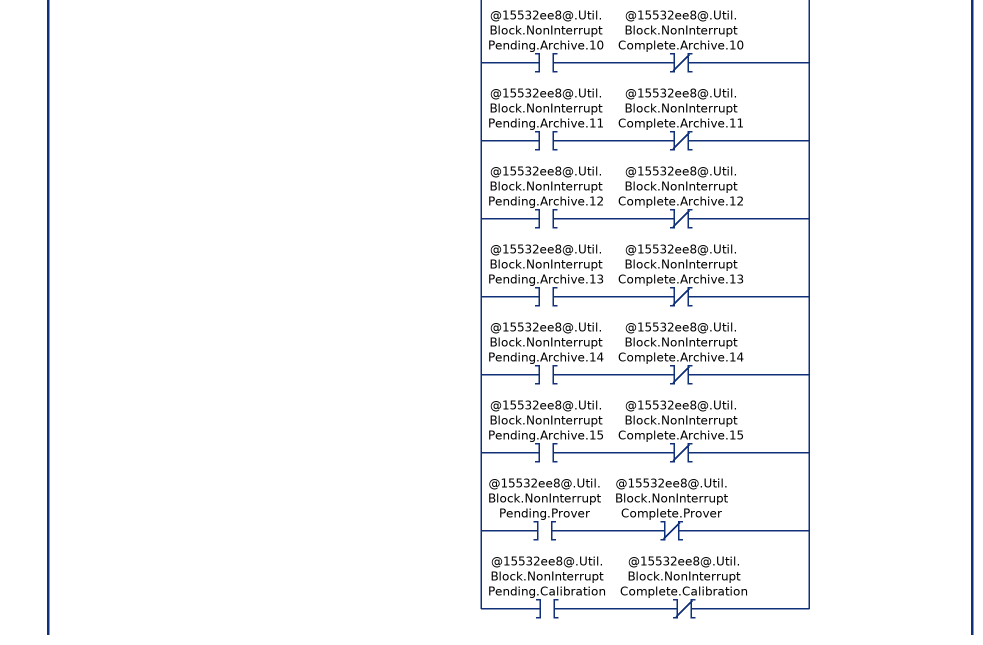
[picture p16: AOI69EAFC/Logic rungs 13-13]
   // Non-Interrupt blocks (1000, 2000 and 5000) occur after Process Input block 12.
   // Check if any non-interrupt block is pending.
   13: XIC(@15532ee8@.Util.Flags.AFCStopped)EQU(@15532ee8@.Util.Buffer.Input[0],12)[XIC(@15532ee8@.Util.Block.NonInterruptPending.ModbusMasterCommand) XIO(@15532ee8@.Util.Block.NonInterruptComplete.ModbusMasterCommand) ,XIC(@15532ee8@.Util.Block.NonInterruptPending.ModbusMasterResponse) XIO(@15532ee8@.Util.Block.NonInterruptComplete.ModbusMasterResponse) ,XIC(@15532ee8@.Util.Block.NonInterruptPending.PassThru) XIO(@15532ee8@.Util.Block.NonInterruptComplete.PassThru) ,XIC(@15532ee8@.Util.Block.NonInterruptPending.Archive.0) XIO(@15532ee8@.Util.Block.NonInterruptComplete.Archive.0) ,XIC(@15532ee8@.Util.Block.NonInterruptPending.Archive.1) XIO(@15532ee8@.Util.Block.NonInterruptComplete.Archive.1) ,XIC(@15532ee8@.Util.Block.NonInterruptPending.Archive.2) XIO(@15532ee8@.Util.Block.NonInterruptComplete.Archive.2) ,XIC(@15532ee8@.Util.Block.NonInterruptPending.Archive.3) XIO(@15532ee8@.Util.Block.NonInterruptComplete.Archive.3) ,XIC(@15532ee8@.Util.Block.NonInterruptPending.Archive.4) XIO(@15532ee8@.Util.Block.NonInterruptComplete.Archive.4) ,XIC(@15532ee8@.Util.Block.NonInterruptPending.Archive.5) XIO(@15532ee8@.Util.Block.NonInterruptComplete.Archive.5) ,XIC(@15532ee8@.Util.Block.NonInterruptPending.Archive.6) XIO(@15532ee8@.Util.Block.NonInterruptComplete.Archive.6) ,XIC(@15532ee8@.Util.Block.NonInterruptPending.Archive.7) XIO(@15532ee8@.Util.Block.NonInterruptComplete.Archive.7) ,XIC(@15532ee8@.Util.Block.NonInterruptPending.Archive.8) XIO(@15532ee8@.Util.Block.NonInterruptComplete.Archive.8) ,XIC(@15532ee8@.Util.Block.NonInterruptPending.Archive.9) XIO(@15532ee8@.Util.Block.NonInterruptComplete.Archive.9) ,XIC(@15532ee8@.Util.Block.NonInterruptPending.Archive.10) XIO(@15532ee8@.Util.Block.NonInterruptComplete.Archive.10) ,XIC(@15532ee8@.Util.Block.NonInterruptPending.Archive.11) XIO(@15532ee8@.Util.Block.NonInterruptComplete.Archive.11) ,XIC(@15532ee8@.Util.Block.NonInterruptPending.Archive.12) XIO(@15532ee8@.Util.Block.NonInterruptComplete.Archive.12) ,XIC(@15532ee8@.Util.Block.NonInterruptPending.Archive.13) XIO(@15532ee8@.Util.Block.NonInterruptComplete.Archive.13) ,XIC(@15532ee8@.Util.Block.NonInterruptPending.Archive.14) XIO(@15532ee8@.Util.Block.NonInterruptComplete.Archive.14) ,XIC(@15532ee8@.Util.Block.NonInterruptPending.Archive.15) XIO(@15532ee8@.Util.Block.NonInterruptComplete.Archive.15) ,XIC(@15532ee8@.Util.Block.NonInterruptPending.Prover) XIO(@15532ee8@.Util.Block.NonInterruptComplete.Prover) ,XIC(@15532ee8@.Util.Block.NonInterruptPending.Calibration) XIO(@15532ee8@.Util.Block.NonInterruptComplete.Calibration) ]OTL(@15532ee8@.Util.Block.NonInterruptPending.Now);
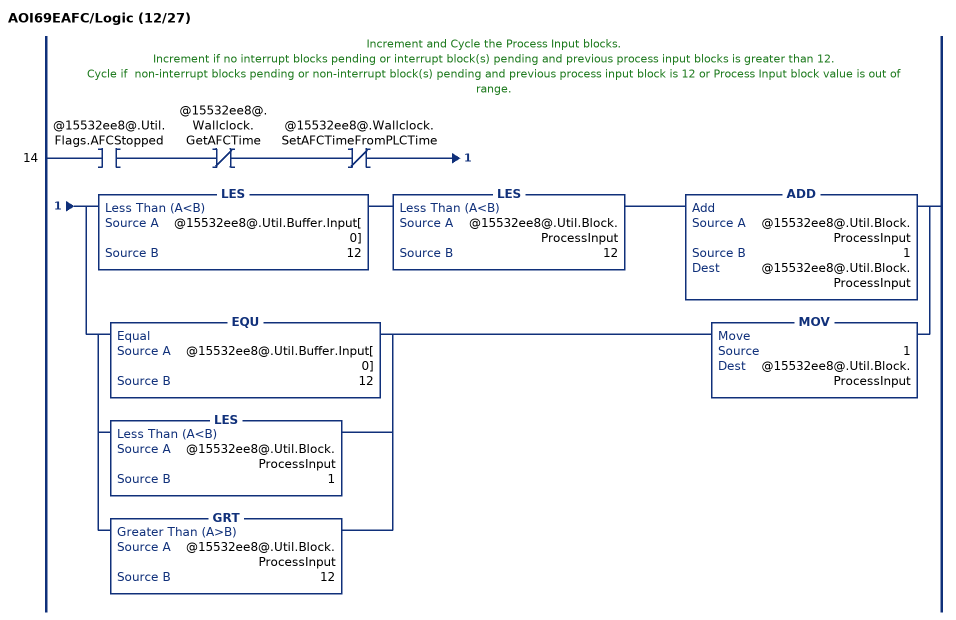
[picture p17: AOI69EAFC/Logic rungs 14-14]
   // Increment and Cycle the Process Input blocks.
   // Increment if no interrupt blocks pending or interrupt block(s) pending and previous process input blocks is greater than 12.
   // Cycle if  non-interrupt blocks pending or non-interrupt block(s) pending and previous process input block is 12 or Process Input block value is out of range.
   14: XIC(@15532ee8@.Util.Flags.AFCStopped)XIO(@15532ee8@.Wallclock.GetAFCTime)XIO(@15532ee8@.Wallclock.SetAFCTimeFromPLCTime)[LES(@15532ee8@.Util.Buffer.Input[0],12) LES(@15532ee8@.Util.Block.ProcessInput,12) ADD(@15532ee8@.Util.Block.ProcessInput,1,@15532ee8@.Util.Block.ProcessInput) ,[EQU(@15532ee8@.Util.Buffer.Input[0],12) ,LES(@15532ee8@.Util.Block.ProcessInput,1) ,GRT(@15532ee8@.Util.Block.ProcessInput,12) ] MOV(1,@15532ee8@.Util.Block.ProcessInput) ];
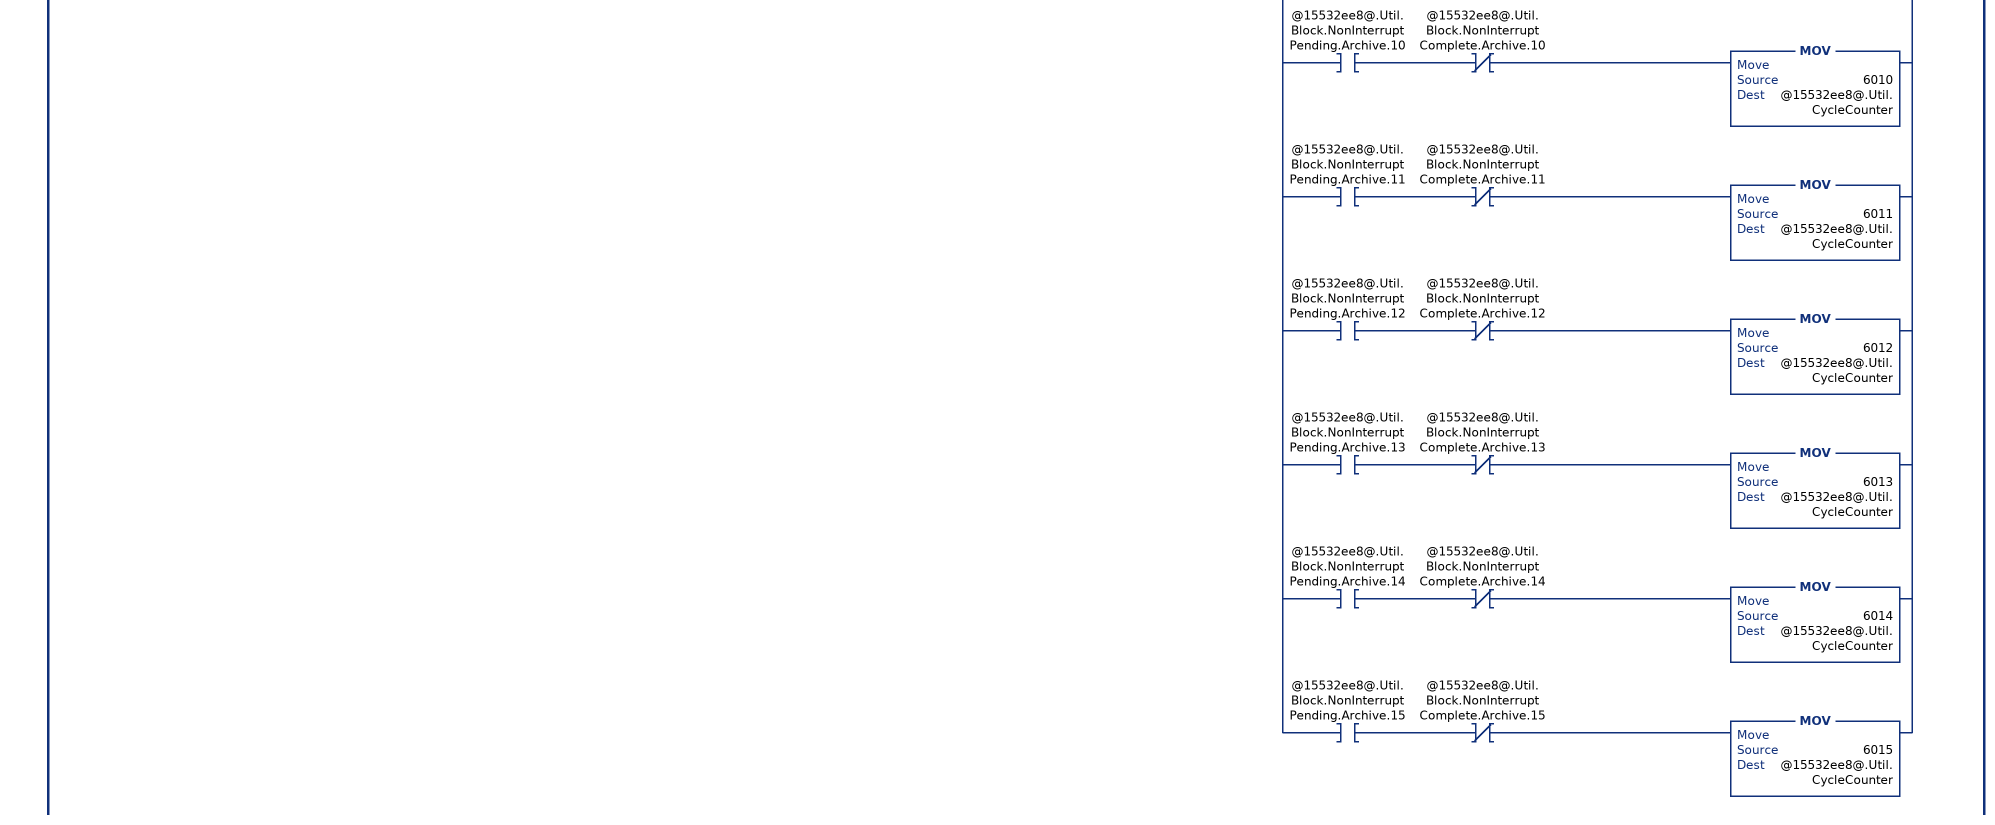
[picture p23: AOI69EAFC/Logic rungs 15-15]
   // Determine the next block to send to module.
   // Send Process Input block if previous block is interrupt or non-interrupt block or either block type is not pending.
   // Send Interrupt block if previous block is Process Input block 1-11 and interrupt block pending.
   // Send Non-interrupt block if previous block is Process Input block 12 and non-interrupt block pending.
   // Note: the block ID has no meaning to the AFC module. The module only requires that the ID changes.
   15: XIC(@15532ee8@.Util.Flags.AFCStopped)XIO(@15532ee8@.Wallclock.GetAFCTime)XIO(@15532ee8@.Wallclock.SetAFCTimeFromPLCTime)[[XIO(@15532ee8@.Util.Block.InterruptPending.Now) LIM(1,@15532ee8@.Util.Buffer.Input[0],11) ,XIO(@15532ee8@.Util.Block.NonInterruptPending.Now) EQU(@15532ee8@.Util.Buffer.Input[0],12) ,GRT(@15532ee8@.Util.Buffer.Input[0],12) ] MOV(@15532ee8@.Util.Block.ProcessInput,@15532ee8@.Util.CycleCounter) ,XIC(@15532ee8@.Util.Block.InterruptPending.Now) LIM(1,@15532ee8@.Util.Buffer.Input[0],11) [[XIC(@15532ee8@.Util.Block.InterruptPending.ModbusGateway.0) XIO(@15532ee8@.Util.Block.InterruptComplete.ModbusGateway.0) MOV(4000,@15532ee8@.Util.CycleCounter) ,XIC(@15532ee8@.Util.Block.InterruptPending.ModbusGateway.1) XIO(@15532ee8@.Util.Block.InterruptComplete.ModbusGateway.1) MOV(4001,@15532ee8@.Util.CycleCounter) ,XIC(@15532ee8@.Util.Block.InterruptPending.ModbusGateway.2) XIO(@15532ee8@.Util.Block.InterruptComplete.ModbusGateway.2) MOV(4002,@15532ee8@.Util.CycleCounter) ,XIC(@15532ee8@.Util.Block.InterruptPending.ModbusGateway.3) XIO(@15532ee8@.Util.Block.InterruptComplete.ModbusGateway.3) MOV(4003,@15532ee8@.Util.CycleCounter) ,XIC(@15532ee8@.Util.Block.InterruptPending.ModbusGateway.4) XIO(@15532ee8@.Util.Block.InterruptComplete.ModbusGateway.4) MOV(4004,@15532ee8@.Util.CycleCounter) ,XIC(@15532ee8@.Util.Block.InterruptPending.ModbusGateway.5) XIO(@15532ee8@.Util.Block.InterruptComplete.ModbusGateway.5) MOV(4005,@15532ee8@.Util.CycleCounter) ,XIC(@15532ee8@.Util.Block.InterruptPending.ModbusGateway.6) XIO(@15532ee8@.Util.Block.InterruptComplete.ModbusGateway.6) MOV(4006,@15532ee8@.Util.CycleCounter) ,XIC(@15532ee8@.Util.Block.InterruptPending.ModbusGateway.7) XIO(@15532ee8@.Util.Block.InterruptComplete.ModbusGateway.7) MOV(4007,@15532ee8@.Util.CycleCounter) ,XIC(@15532ee8@.Util.Block.InterruptPending.ModbusGateway.8) XIO(@15532ee8@.Util.Block.InterruptComplete.ModbusGateway.8) MOV(4008,@15532ee8@.Util.CycleCounter) ,XIC(@15532ee8@.Util.Block.InterruptPending.ModbusGateway.9) XIO(@15532ee8@.Util.Block.InterruptComplete.ModbusGateway.9) MOV(4009,@15532ee8@.Util.CycleCounter) ] ,EQU(@15532ee8@.Util.Block.InterruptPending.ModbusGateway,0) XIC(@15532ee8@.Util.Block.InterruptPending.EnableDisable) XIO(@15532ee8@.Util.Block.InterruptComplete.EnableDisable) MOV(7000,@15532ee8@.Util.CycleCounter) ,EQU(@15532ee8@.Util.Block.InterruptPending.ModbusGateway,0) XIO(@15532ee8@.Util.Block.InterruptPending.EnableDisable) [XIC(@15532ee8@.Util.Block.InterruptPending.Analysis.0) XIO(@15532ee8@.Util.Block.InterruptComplete.Analysis.0) MOV(3000,@15532ee8@.Util.CycleCounter) ,XIC(@15532ee8@.Util.Block.InterruptPending.Analysis.1) XIO(@15532ee8@.Util.Block.InterruptComplete.Analysis.1) MOV(3001,@15532ee8@.Util.CycleCounter) ,XIC(@15532ee8@.Util.Block.InterruptPending.Analysis.2) XIO(@15532ee8@.Util.Block.InterruptComplete.Analysis.2) MOV(3002,@15532ee8@.Util.CycleCounter) ,XIC(@15532ee8@.Util.Block.InterruptPending.Analysis.3) XIO(@15532ee8@.Util.Block.InterruptComplete.Analysis.3) MOV(3003,@15532ee8@.Util.CycleCounter) ,XIC(@15532ee8@.Util.Block.InterruptPending.Analysis.4) XIO(@15532ee8@.Util.Block.InterruptComplete.Analysis.4) MOV(3004,@15532ee8@.Util.CycleCounter) ,XIC(@15532ee8@.Util.Block.InterruptPending.Analysis.5) XIO(@15532ee8@.Util.Block.InterruptComplete.Analysis.5) MOV(3005,@15532ee8@.Util.CycleCounter) ] ] ,XIC(@15532ee8@.Util.Block.NonInterruptPending.Now) EQU(@15532ee8@.Util.Buffer.Input[0],12) [XIC(@15532ee8@.ModbusMaster.Enable) LIM(0,@15532ee8@.ModbusMaster.CommandIndex,9) [XIO(@15532ee8@.Util.Block.NonInterruptComplete.ModbusMasterCommand) XIC(@15532ee8@.ModbusMaster.Command[@15532ee8@.ModbusMaster.CommandIndex].Config.Enable) XIO(@15532ee8@.SiteStatus.ModbusMasterPending) XIO(@15532ee8@.SiteStatus.ModbusMasterComplete) MOV(1000,@15532ee8@.Util.CycleCounter) ,XIO(@15532ee8@.Util.Block.NonInterruptComplete.ModbusMasterResponse) XIC(@15532ee8@.SiteStatus.ModbusMasterComplete) MOV(1001,@15532ee8@.Util.CycleCounter) ] ,XIO(@15532ee8@.Util.Block.NonInterruptPending.ModbusMasterCommand) XIO(@15532ee8@.Util.Block.NonInterruptPending.ModbusMasterResponse) [XIC(@15532ee8@.ModbusPassThru.Enable) XIC(@15532ee8@.SiteStatus.ModbusPassThruPending) XIC(@15532ee8@.ModbusPassThru.GetMessage) MOV(2000,@15532ee8@.Util.CycleCounter) ,XIO(@15532ee8@.Util.Block.NonInterruptPending.PassThru) [XIC(@15532ee8@.Util.Block.NonInterruptPending.Prover) XIO(@15532ee8@.Util.Block.NonInterruptComplete.Prover) XIC(@15532ee8@.Prove.ProveEnabled) MOV(5000,@15532ee8@.Util.CycleCounter) ,XIO(@15532ee8@.Util.Block.NonInterruptPending.Prover) [XIC(@15532ee8@.SiteStatus.CalibrationRequest) XIO(@15532ee8@.Util.Block.NonInterruptComplete.Calibration) [EQU(@15532ee8@.Util.Buffer.Calibration[1],0) MOV(9000,@15532ee8@.Util.CycleCounter) ,NEQ(@15532ee8@.Util.Buffer.Calibration[1],0) MOV(9001,@15532ee8@.Util.CycleCounter) ] ,XIO(@15532ee8@.Util.Block.NonInterruptPending.Calibration) [XIC(@15532ee8@.Util.Block.NonInterruptPending.Archive.0) XIO(@15532ee8@.Util.Block.NonInterruptComplete.Archive.0) MOV(6000,@15532ee8@.Util.CycleCounter) ,XIC(@15532ee8@.Util.Block.NonInterruptPending.Archive.1) XIO(@15532ee8@.Util.Block.NonInterruptComplete.Archive.1) MOV(6001,@15532ee8@.Util.CycleCounter) ,XIC(@15532ee8@.Util.Block.NonInterruptPending.Archive.2) XIO(@15532ee8@.Util.Block.NonInterruptComplete.Archive.2) MOV(6002,@15532ee8@.Util.CycleCounter) ,XIC(@15532ee8@.Util.Block.NonInterruptPending.Archive.3) XIO(@15532ee8@.Util.Block.NonInterruptComplete.Archive.3) MOV(6003,@15532ee8@.Util.CycleCounter) ,XIC(@15532ee8@.Util.Block.NonInterruptPending.Archive.4) XIO(@15532ee8@.Util.Block.NonInterruptComplete.Archive.4) MOV(6004,@15532ee8@.Util.CycleCounter) ,XIC(@15532ee8@.Util.Block.NonInterruptPending.Archive.5) XIO(@15532ee8@.Util.Block.NonInterruptComplete.Archive.5) MOV(6005,@15532ee8@.Util.CycleCounter) ,XIC(@15532ee8@.Util.Block.NonInterruptPending.Archive.6) XIO(@15532ee8@.Util.Block.NonInterruptComplete.Archive.6) MOV(6006,@15532ee8@.Util.CycleCounter) ,XIC(@15532ee8@.Util.Block.NonInterruptPending.Archive.7) XIO(@15532ee8@.Util.Block.NonInterruptComplete.Archive.7) MOV(6007,@15532ee8@.Util.CycleCounter) ,XIC(@15532ee8@.Util.Block.NonInterruptPending.Archive.8) XIO(@15532ee8@.Util.Block.NonInterruptComplete.Archive.8) MOV(6008,@15532ee8@.Util.CycleCounter) ,XIC(@15532ee8@.Util.Block.NonInterruptPending.Archive.9) XIO(@15532ee8@.Util.Block.NonInterruptComplete.Archive.9) MOV(6009,@15532ee8@.Util.CycleCounter) ,XIC(@15532ee8@.Util.Block.NonInterruptPending.Archive.10) XIO(@15532ee8@.Util.Block.NonInterruptComplete.Archive.10) MOV(6010,@15532ee8@.Util.CycleCounter) ,XIC(@15532ee8@.Util.Block.NonInterruptPending.Archive.11) XIO(@15532ee8@.Util.Block.NonInterruptComplete.Archive.11) MOV(6011,@15532ee8@.Util.CycleCounter) ,XIC(@15532ee8@.Util.Block.NonInterruptPending.Archive.12) XIO(@15532ee8@.Util.Block.NonInterruptComplete.Archive.12) MOV(6012,@15532ee8@.Util.CycleCounter) ,XIC(@15532ee8@.Util.Block.NonInterruptPending.Archive.13) XIO(@15532ee8@.Util.Block.NonInterruptComplete.Archive.13) MOV(6013,@15532ee8@.Util.CycleCounter) ,XIC(@15532ee8@.Util.Block.NonInterruptPending.Archive.14) XIO(@15532ee8@.Util.Block.NonInterruptComplete.Archive.14) MOV(6014,@15532ee8@.Util.CycleCounter) ,XIC(@15532ee8@.Util.Block.NonInterruptPending.Archive.15) XIO(@15532ee8@.Util.Block.NonInterruptComplete.Archive.15) MOV(6015,@15532ee8@.Util.CycleCounter) ] ] ] ] ] ];
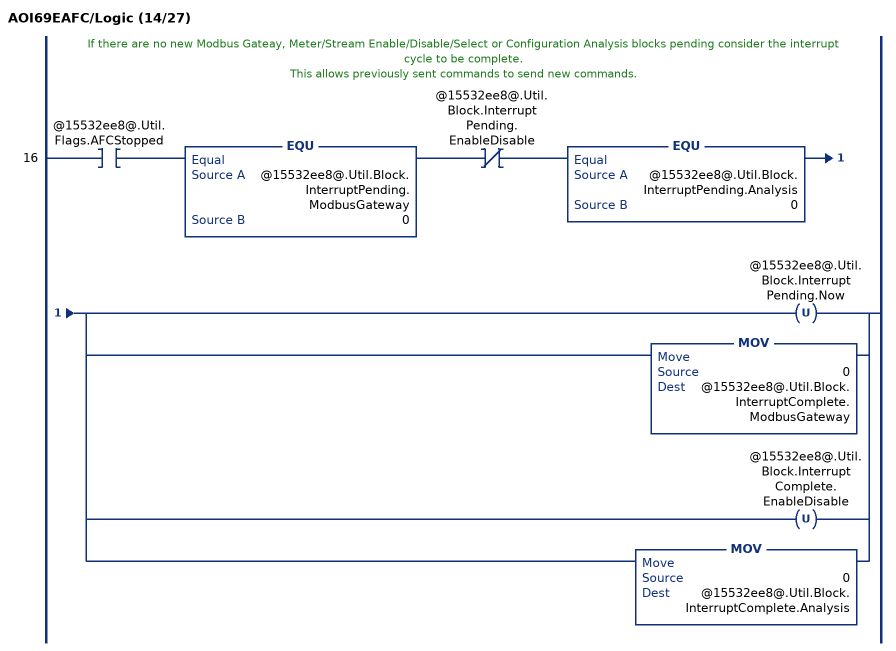
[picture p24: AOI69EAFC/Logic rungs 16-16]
   // If there are no new Modbus Gateay, Meter/Stream Enable/Disable/Select or Configuration Analysis blocks pending consider the interrupt cycle to be complete.
   // This allows previously sent commands to send new commands.
   16: XIC(@15532ee8@.Util.Flags.AFCStopped)EQU(@15532ee8@.Util.Block.InterruptPending.ModbusGateway,0)XIO(@15532ee8@.Util.Block.InterruptPending.EnableDisable)EQU(@15532ee8@.Util.Block.InterruptPending.Analysis,0)[OTU(@15532ee8@.Util.Block.InterruptPending.Now) ,MOV(0,@15532ee8@.Util.Block.InterruptComplete.ModbusGateway) ,OTU(@15532ee8@.Util.Block.InterruptComplete.EnableDisable) ,MOV(0,@15532ee8@.Util.Block.InterruptComplete.Analysis) ];
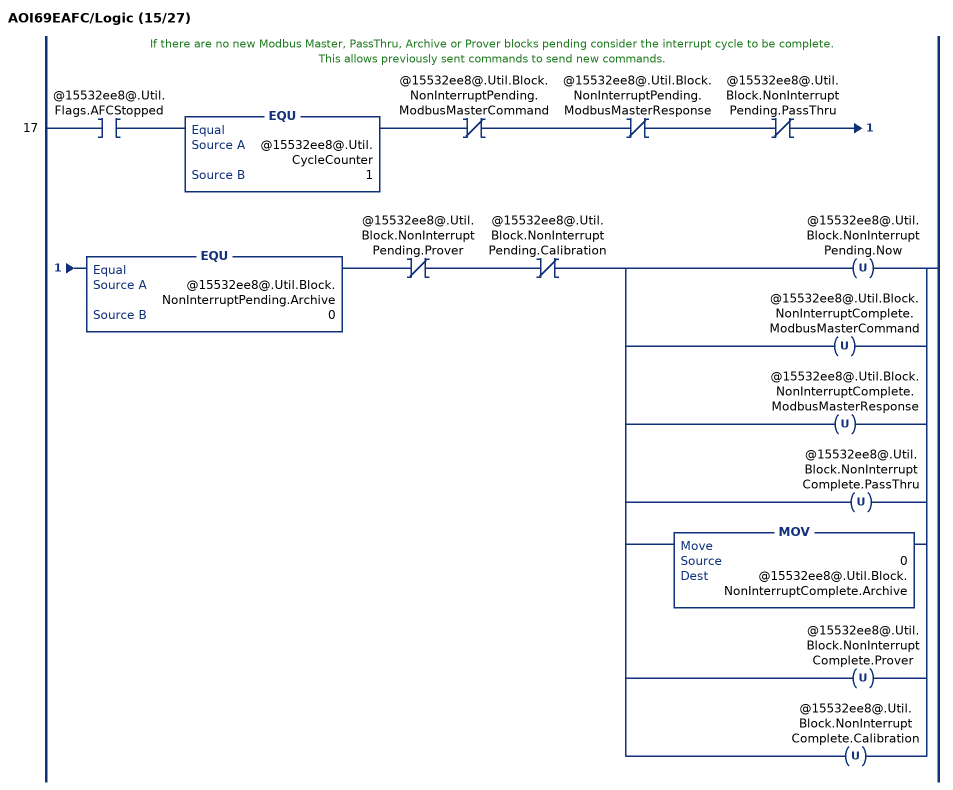
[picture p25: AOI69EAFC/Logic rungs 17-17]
   // If there are no new Modbus Master, PassThru, Archive or Prover blocks pending consider the interrupt cycle to be complete.
   // This allows previously sent commands to send new commands.
   17: XIC(@15532ee8@.Util.Flags.AFCStopped)EQU(@15532ee8@.Util.CycleCounter,1)XIO(@15532ee8@.Util.Block.NonInterruptPending.ModbusMasterCommand)XIO(@15532ee8@.Util.Block.NonInterruptPending.ModbusMasterResponse)XIO(@15532ee8@.Util.Block.NonInterruptPending.PassThru)EQU(@15532ee8@.Util.Block.NonInterruptPending.Archive,0)XIO(@15532ee8@.Util.Block.NonInterruptPending.Prover)XIO(@15532ee8@.Util.Block.NonInterruptPending.Calibration)[OTU(@15532ee8@.Util.Block.NonInterruptPending.Now) ,OTU(@15532ee8@.Util.Block.NonInterruptComplete.ModbusMasterCommand) ,OTU(@15532ee8@.Util.Block.NonInterruptComplete.ModbusMasterResponse) ,OTU(@15532ee8@.Util.Block.NonInterruptComplete.PassThru) ,MOV(0,@15532ee8@.Util.Block.NonInterruptComplete.Archive) ,OTU(@15532ee8@.Util.Block.NonInterruptComplete.Prover) ,OTU(@15532ee8@.Util.Block.NonInterruptComplete.Calibration) ];
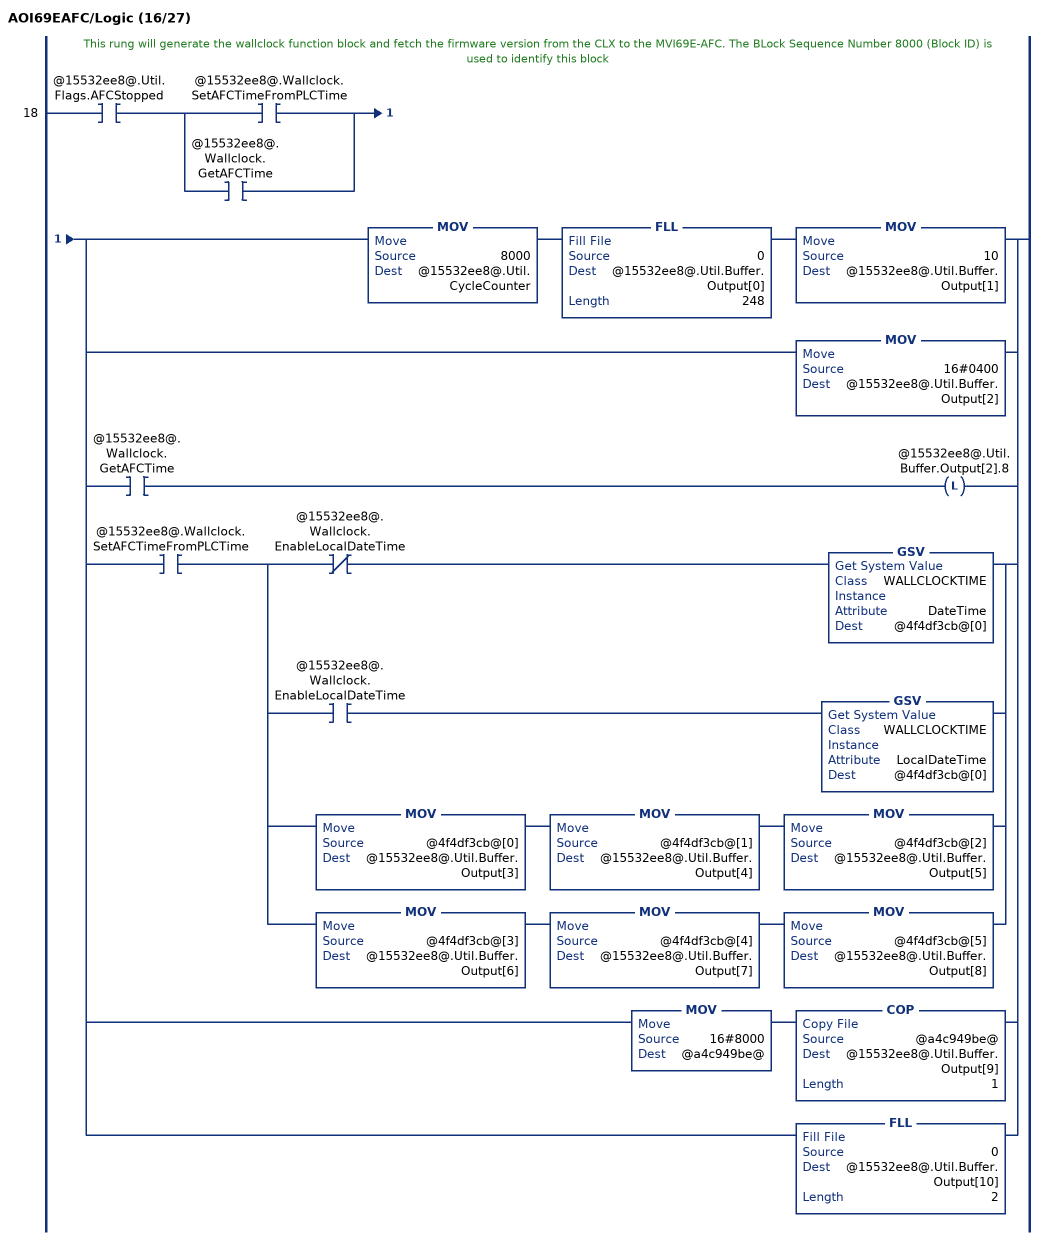
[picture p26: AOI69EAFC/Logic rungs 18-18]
   // This rung will generate the wallclock function block and fetch the firmware version from the CLX to the MVI69E-AFC. The BLock Sequence Number 8000 (Block ID) is used to identify this block
   18: XIC(@15532ee8@.Util.Flags.AFCStopped)[XIC(@15532ee8@.Wallclock.SetAFCTimeFromPLCTime) ,XIC(@15532ee8@.Wallclock.GetAFCTime) ][MOV(8000,@15532ee8@.Util.CycleCounter) FLL(0,@15532ee8@.Util.Buffer.Output[0],248) MOV(10,@15532ee8@.Util.Buffer.Output[1]) ,[MOV(16#0400,@15532ee8@.Util.Buffer.Output[2]) ,XIC(@15532ee8@.Wallclock.GetAFCTime) OTL(@15532ee8@.Util.Buffer.Output[2].8) ] ,XIC(@15532ee8@.Wallclock.SetAFCTimeFromPLCTime) [[XIO(@15532ee8@.Wallclock.EnableLocalDateTime) GSV(WALLCLOCKTIME,,DateTime,@4f4df3cb@[0]) ,XIC(@15532ee8@.Wallclock.EnableLocalDateTime) GSV(WALLCLOCKTIME,,LocalDateTime,@4f4df3cb@[0]) ] ,MOV(@4f4df3cb@[0],@15532ee8@.Util.Buffer.Output[3]) MOV(@4f4df3cb@[1],@15532ee8@.Util.Buffer.Output[4]) MOV(@4f4df3cb@[2],@15532ee8@.Util.Buffer.Output[5]) ,MOV(@4f4df3cb@[3],@15532ee8@.Util.Buffer.Output[6]) MOV(@4f4df3cb@[4],@15532ee8@.Util.Buffer.Output[7]) MOV(@4f4df3cb@[5],@15532ee8@.Util.Buffer.Output[8]) ] ,[MOV(16#8000,@a4c949be@) COP(@a4c949be@,@15532ee8@.Util.Buffer.Output[9],1) ,FLL(0,@15532ee8@.Util.Buffer.Output[10],2) ] ];
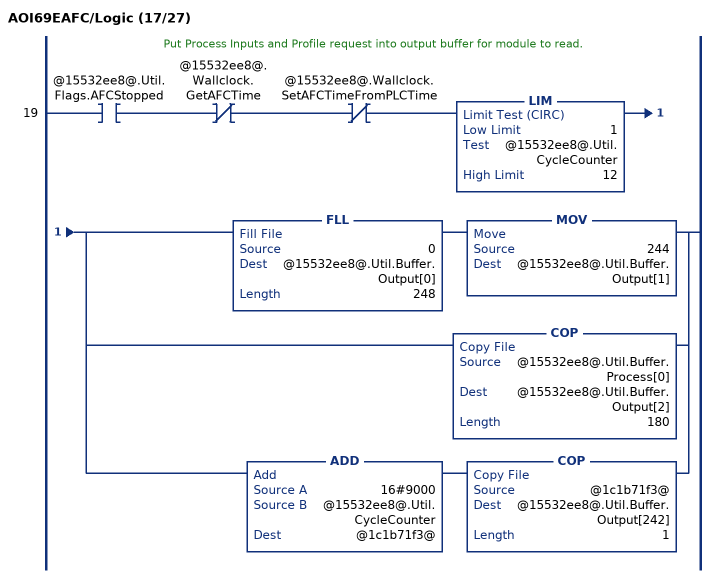
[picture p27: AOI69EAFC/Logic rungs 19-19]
   // Put Process Inputs and Profile request into output buffer for module to read.
   19: XIC(@15532ee8@.Util.Flags.AFCStopped)XIO(@15532ee8@.Wallclock.GetAFCTime)XIO(@15532ee8@.Wallclock.SetAFCTimeFromPLCTime)LIM(1,@15532ee8@.Util.CycleCounter,12)[FLL(0,@15532ee8@.Util.Buffer.Output[0],248) MOV(244,@15532ee8@.Util.Buffer.Output[1]) ,COP(@15532ee8@.Util.Buffer.Process[0],@15532ee8@.Util.Buffer.Output[2],180) ,ADD(16#9000,@15532ee8@.Util.CycleCounter,@1c1b71f3@) COP(@1c1b71f3@,@15532ee8@.Util.Buffer.Output[242],1) ];
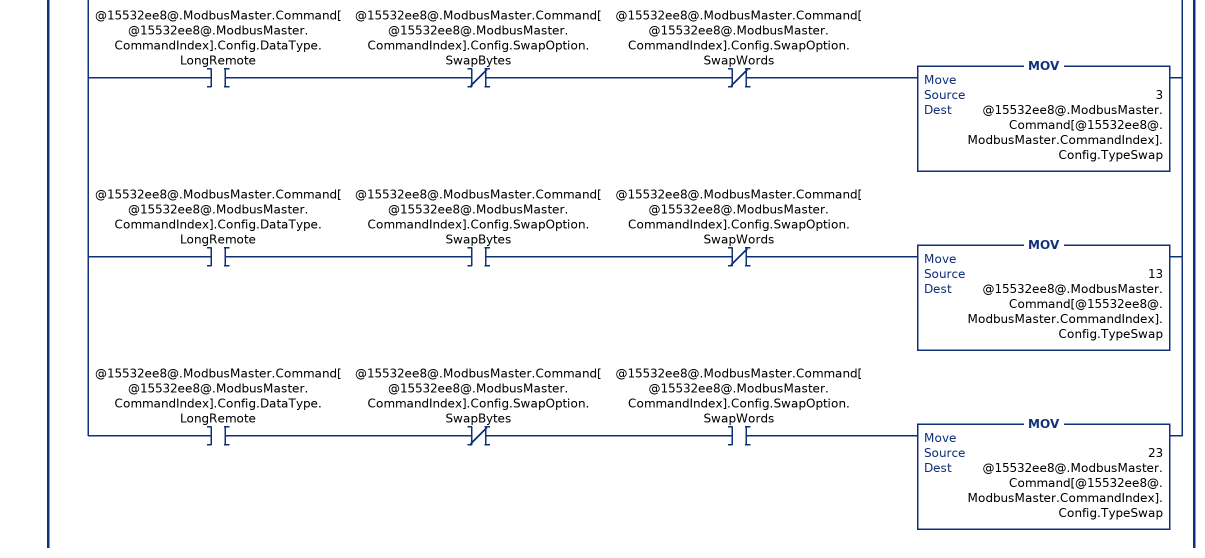
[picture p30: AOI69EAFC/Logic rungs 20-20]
   // Setup Modbus Master command.
   20: XIC(@15532ee8@.Util.Flags.AFCStopped)XIO(@15532ee8@.Wallclock.GetAFCTime)XIO(@15532ee8@.Wallclock.SetAFCTimeFromPLCTime)XIC(@15532ee8@.ModbusMaster.Enable)LIM(0,@15532ee8@.ModbusMaster.CommandIndex,9)[EQU(@15532ee8@.Util.CycleCounter,1000) XIO(@15532ee8@.Util.Block.NonInterruptComplete.ModbusMasterCommand) ,EQU(@15532ee8@.Util.CycleCounter,1001) XIO(@15532ee8@.Util.Block.NonInterruptComplete.ModbusMasterResponse) ][ADD(16#6000,130,@7a00ef8d@) ,[XIC(@15532ee8@.ModbusMaster.Command[@15532ee8@.ModbusMaster.CommandIndex].Config.FunctionType) [OTE(@7a00ef8d@.11) ,OTL(@13d1991b@) ] ,XIO(@15532ee8@.ModbusMaster.Command[@15532ee8@.ModbusMaster.CommandIndex].Config.FunctionType) OTU(@13d1991b@) ] ,XIO(@15532ee8@.ModbusMaster.Command[@15532ee8@.ModbusMaster.CommandIndex].Config.Enable) OTE(@7a00ef8d@.8) ,XIC(@15532ee8@.ModbusMaster.Command[@15532ee8@.ModbusMaster.CommandIndex].Config.RegisterBank) OTE(@7a00ef8d@.10) ,XIC(@15532ee8@.ModbusMaster.Command[@15532ee8@.ModbusMaster.CommandIndex].Config.DataType.Bit) MOV(0,@15532ee8@.ModbusMaster.Command[@15532ee8@.ModbusMaster.CommandIndex].Config.TypeSwap) ,XIC(@15532ee8@.ModbusMaster.Command[@15532ee8@.ModbusMaster.CommandIndex].Config.DataType.Word) XIO(@15532ee8@.ModbusMaster.Command[@15532ee8@.ModbusMaster.CommandIndex].Config.SwapOption.SwapBytes) MOV(1,@15532ee8@.ModbusMaster.Command[@15532ee8@.ModbusMaster.CommandIndex].Config.TypeSwap) ,XIC(@15532ee8@.ModbusMaster.Command[@15532ee8@.ModbusMaster.CommandIndex].Config.DataType.Word) XIC(@15532ee8@.ModbusMaster.Command[@15532ee8@.ModbusMaster.CommandIndex].Config.SwapOption.SwapBytes) MOV(11,@15532ee8@.ModbusMaster.Command[@15532ee8@.ModbusMaster.CommandIndex].Config.TypeSwap) ,XIC(@15532ee8@.ModbusMaster.Command[@15532ee8@.ModbusMaster.CommandIndex].Config.DataType.Long) XIO(@15532ee8@.ModbusMaster.Command[@15532ee8@.ModbusMaster.CommandIndex].Config.SwapOption.SwapBytes) XIO(@15532ee8@.ModbusMaster.Command[@15532ee8@.ModbusMaster.CommandIndex].Config.SwapOption.SwapWords) MOV(2,@15532ee8@.ModbusMaster.Command[@15532ee8@.ModbusMaster.CommandIndex].Config.TypeSwap) ,XIC(@15532ee8@.ModbusMaster.Command[@15532ee8@.ModbusMaster.CommandIndex].Config.DataType.Long) XIC(@15532ee8@.ModbusMaster.Command[@15532ee8@.ModbusMaster.CommandIndex].Config.SwapOption.SwapBytes) XIO(@15532ee8@.ModbusMaster.Command[@15532ee8@.ModbusMaster.CommandIndex].Config.SwapOption.SwapWords) MOV(12,@15532ee8@.ModbusMaster.Command[@15532ee8@.ModbusMaster.CommandIndex].Config.TypeSwap) ,XIC(@15532ee8@.ModbusMaster.Command[@15532ee8@.ModbusMaster.CommandIndex].Config.DataType.Long) XIO(@15532ee8@.ModbusMaster.Command[@15532ee8@.ModbusMaster.CommandIndex].Config.SwapOption.SwapBytes) XIC(@15532ee8@.ModbusMaster.Command[@15532ee8@.ModbusMaster.CommandIndex].Config.SwapOption.SwapWords) MOV(22,@15532ee8@.ModbusMaster.Command[@15532ee8@.ModbusMaster.CommandIndex].Config.TypeSwap) ,XIC(@15532ee8@.ModbusMaster.Command[@15532ee8@.ModbusMaster.CommandIndex].Config.DataType.LongRemote) XIO(@15532ee8@.ModbusMaster.Command[@15532ee8@.ModbusMaster.CommandIndex].Config.SwapOption.SwapBytes) XIO(@15532ee8@.ModbusMaster.Command[@15532ee8@.ModbusMaster.CommandIndex].Config.SwapOption.SwapWords) MOV(3,@15532ee8@.ModbusMaster.Command[@15532ee8@.ModbusMaster.CommandIndex].Config.TypeSwap) ,XIC(@15532ee8@.ModbusMaster.Command[@15532ee8@.ModbusMaster.CommandIndex].Config.DataType.LongRemote) XIC(@15532ee8@.ModbusMaster.Command[@15532ee8@.ModbusMaster.CommandIndex].Config.SwapOption.SwapBytes) XIO(@15532ee8@.ModbusMaster.Command[@15532ee8@.ModbusMaster.CommandIndex].Config.SwapOption.SwapWords) MOV(13,@15532ee8@.ModbusMaster.Command[@15532ee8@.ModbusMaster.CommandIndex].Config.TypeSwap) ,XIC(@15532ee8@.ModbusMaster.Command[@15532ee8@.ModbusMaster.CommandIndex].Config.DataType.LongRemote) XIO(@15532ee8@.ModbusMaster.Command[@15532ee8@.ModbusMaster.CommandIndex].Config.SwapOption.SwapBytes) XIC(@15532ee8@.ModbusMaster.Command[@15532ee8@.ModbusMaster.CommandIndex].Config.SwapOption.SwapWords) MOV(23,@15532ee8@.ModbusMaster.Command[@15532ee8@.ModbusMaster.CommandIndex].Config.TypeSwap) ];
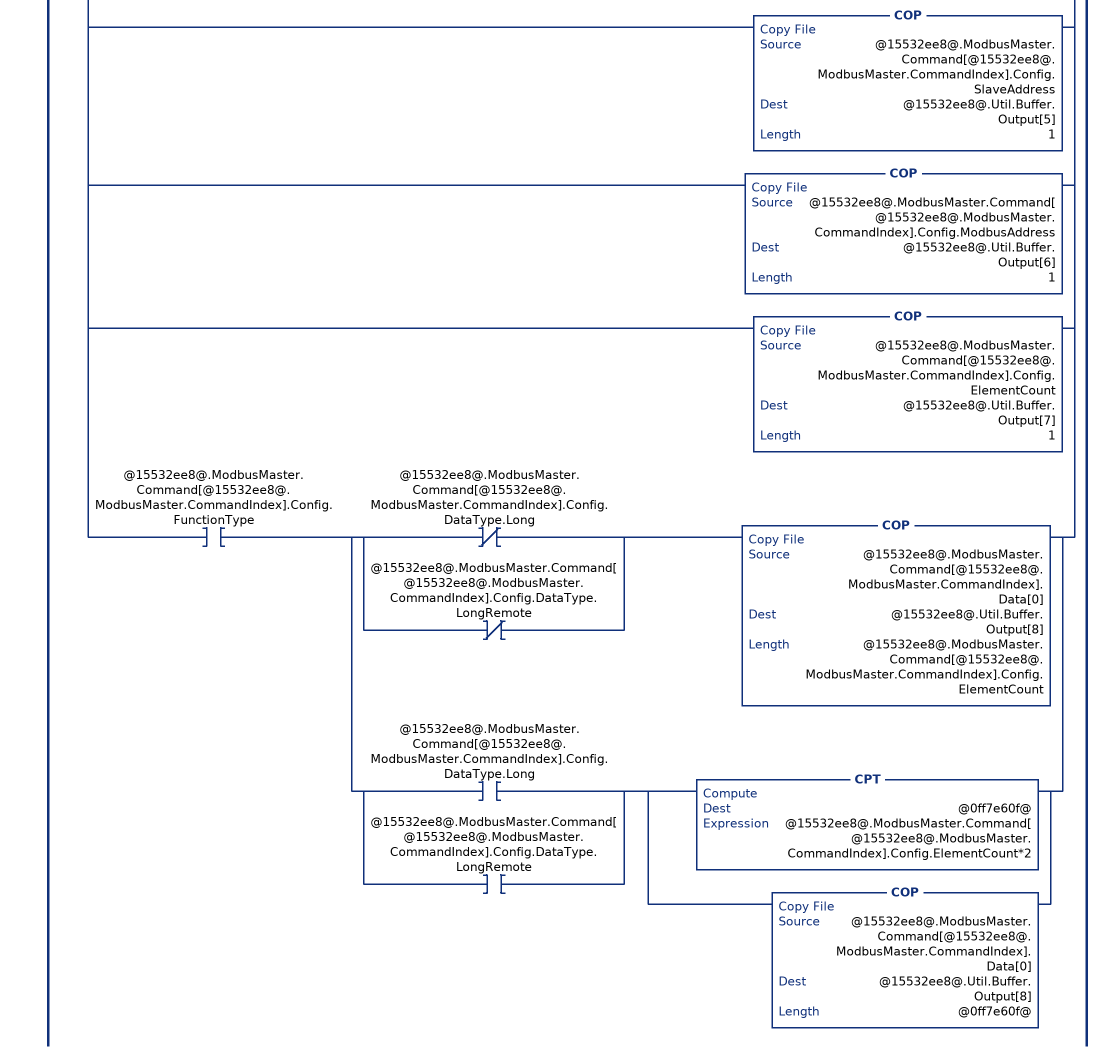
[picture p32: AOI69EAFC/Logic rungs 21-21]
   // Put Modbus Master command into output buffer for module to read.
   21: XIC(@15532ee8@.Util.Flags.AFCStopped)XIO(@15532ee8@.Wallclock.GetAFCTime)XIO(@15532ee8@.Wallclock.SetAFCTimeFromPLCTime)XIC(@15532ee8@.ModbusMaster.Enable)LIM(0,@15532ee8@.ModbusMaster.CommandIndex,9)[EQU(@15532ee8@.Util.CycleCounter,1000) XIO(@15532ee8@.Util.Block.NonInterruptComplete.ModbusMasterCommand) ,EQU(@15532ee8@.Util.CycleCounter,1001) XIO(@15532ee8@.Util.Block.NonInterruptComplete.ModbusMasterResponse) ][MOV(131,@15532ee8@.Util.Buffer.Output[1]) ,COP(@7a00ef8d@,@15532ee8@.Util.Buffer.Output[2],1) ,COP(@15532ee8@.ModbusMaster.Command[@15532ee8@.ModbusMaster.CommandIndex].Config.TransactionID,@15532ee8@.Util.Buffer.Output[3],1) ,COP(@15532ee8@.ModbusMaster.Command[@15532ee8@.ModbusMaster.CommandIndex].Config.TypeSwap,@15532ee8@.Util.Buffer.Output[4],1) ,COP(@15532ee8@.ModbusMaster.Command[@15532ee8@.ModbusMaster.CommandIndex].Config.SlaveAddress,@15532ee8@.Util.Buffer.Output[5],1) ,COP(@15532ee8@.ModbusMaster.Command[@15532ee8@.ModbusMaster.CommandIndex].Config.ModbusAddress,@15532ee8@.Util.Buffer.Output[6],1) ,COP(@15532ee8@.ModbusMaster.Command[@15532ee8@.ModbusMaster.CommandIndex].Config.ElementCount,@15532ee8@.Util.Buffer.Output[7],1) ,XIC(@15532ee8@.ModbusMaster.Command[@15532ee8@.ModbusMaster.CommandIndex].Config.FunctionType) [[XIO(@15532ee8@.ModbusMaster.Command[@15532ee8@.ModbusMaster.CommandIndex].Config.DataType.Long) ,XIO(@15532ee8@.ModbusMaster.Command[@15532ee8@.ModbusMaster.CommandIndex].Config.DataType.LongRemote) ] COP(@15532ee8@.ModbusMaster.Command[@15532ee8@.ModbusMaster.CommandIndex].Data[0],@15532ee8@.Util.Buffer.Output[8],@15532ee8@.ModbusMaster.Command[@15532ee8@.ModbusMaster.CommandIndex].Config.ElementCount) ,[XIC(@15532ee8@.ModbusMaster.Command[@15532ee8@.ModbusMaster.CommandIndex].Config.DataType.Long) ,XIC(@15532ee8@.ModbusMaster.Command[@15532ee8@.ModbusMaster.CommandIndex].Config.DataType.LongRemote) ] [CPT(@0ff7e60f@,@15532ee8@.ModbusMaster.Command[@15532ee8@.ModbusMaster.CommandIndex].Config.ElementCount*2) ,COP(@15532ee8@.ModbusMaster.Command[@15532ee8@.ModbusMaster.CommandIndex].Data[0],@15532ee8@.Util.Buffer.Output[8],@0ff7e60f@) ] ] ];
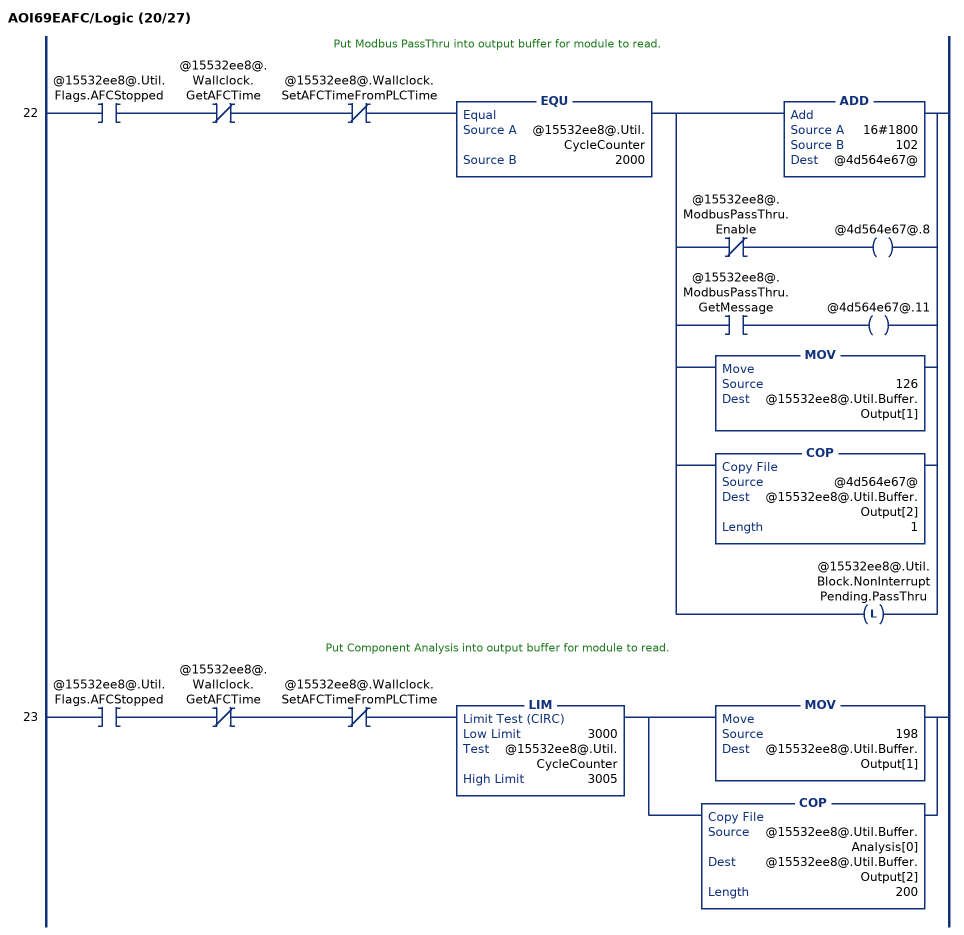
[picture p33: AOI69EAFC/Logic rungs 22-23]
   // Put Modbus PassThru into output buffer for module to read.
   22: XIC(@15532ee8@.Util.Flags.AFCStopped)XIO(@15532ee8@.Wallclock.GetAFCTime)XIO(@15532ee8@.Wallclock.SetAFCTimeFromPLCTime)EQU(@15532ee8@.Util.CycleCounter,2000)[ADD(16#1800,102,@4d564e67@) ,XIO(@15532ee8@.ModbusPassThru.Enable) OTE(@4d564e67@.8) ,XIC(@15532ee8@.ModbusPassThru.GetMessage) OTE(@4d564e67@.11) ,MOV(126,@15532ee8@.Util.Buffer.Output[1]) ,COP(@4d564e67@,@15532ee8@.Util.Buffer.Output[2],1) ,OTL(@15532ee8@.Util.Block.NonInterruptPending.PassThru) ];
   // Put Component Analysis into output buffer for module to read.
   23: XIC(@15532ee8@.Util.Flags.AFCStopped)XIO(@15532ee8@.Wallclock.GetAFCTime)XIO(@15532ee8@.Wallclock.SetAFCTimeFromPLCTime)LIM(3000,@15532ee8@.Util.CycleCounter,3005)[MOV(198,@15532ee8@.Util.Buffer.Output[1]) ,COP(@15532ee8@.Util.Buffer.Analysis[0],@15532ee8@.Util.Buffer.Output[2],200) ];
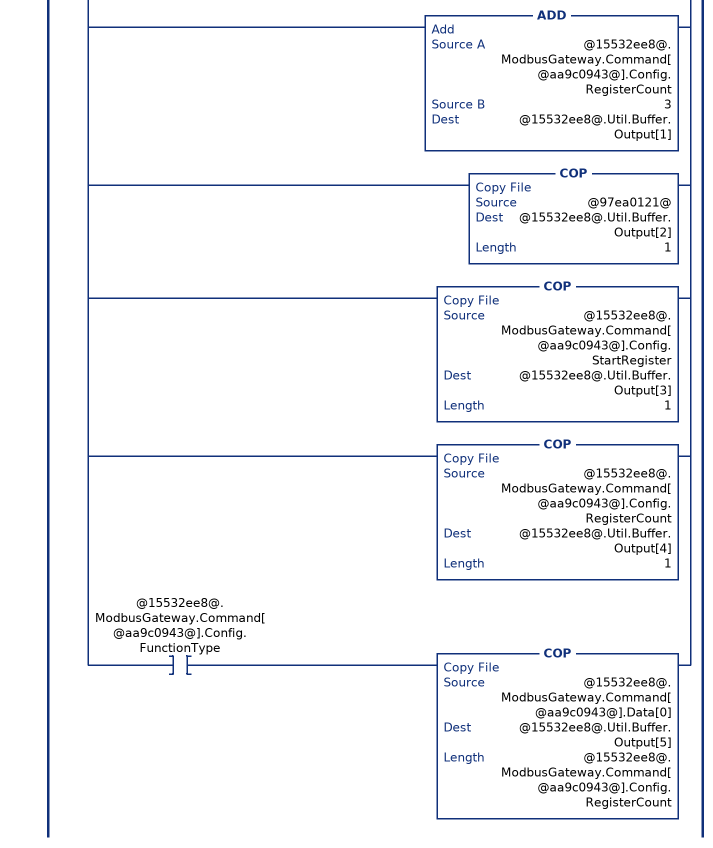
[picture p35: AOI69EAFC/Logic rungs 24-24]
   // Put Modbus Gateway command into output buffer for module to read.
   24: XIC(@15532ee8@.Util.Flags.AFCStopped)XIO(@15532ee8@.Wallclock.GetAFCTime)XIO(@15532ee8@.Wallclock.SetAFCTimeFromPLCTime)LIM(4000,@15532ee8@.Util.CycleCounter,4009)[SUB(@15532ee8@.Util.CycleCounter,4000,@aa9c0943@) CPT(@771d54c0@,2**@aa9c0943@) ,MOV(16#4000,@97ea0121@) ,XIO(@15532ee8@.ModbusGateway.Command[@aa9c0943@].Config.Enable) OTE(@97ea0121@.8) ,XIC(@15532ee8@.ModbusGateway.Command[@aa9c0943@].Config.SlaveType) OTE(@97ea0121@.10) ,XIC(@15532ee8@.ModbusGateway.Command[@aa9c0943@].Config.RegisterType) OTE(@97ea0121@.11) ,XIC(@15532ee8@.ModbusGateway.Command[@aa9c0943@].Config.FunctionType) OTE(@97ea0121@.12) ,CPT(@97ea0121@,@97ea0121@+@15532ee8@.ModbusGateway.Command[@aa9c0943@].Config.RegisterCount+2) ,FLL(0,@15532ee8@.Util.Buffer.Output[1],246) ,ADD(@15532ee8@.ModbusGateway.Command[@aa9c0943@].Config.RegisterCount,3,@15532ee8@.Util.Buffer.Output[1]) ,COP(@97ea0121@,@15532ee8@.Util.Buffer.Output[2],1) ,COP(@15532ee8@.ModbusGateway.Command[@aa9c0943@].Config.StartRegister,@15532ee8@.Util.Buffer.Output[3],1) ,COP(@15532ee8@.ModbusGateway.Command[@aa9c0943@].Config.RegisterCount,@15532ee8@.Util.Buffer.Output[4],1) ,XIC(@15532ee8@.ModbusGateway.Command[@aa9c0943@].Config.FunctionType) COP(@15532ee8@.ModbusGateway.Command[@aa9c0943@].Data[0],@15532ee8@.Util.Buffer.Output[5],@15532ee8@.ModbusGateway.Command[@aa9c0943@].Config.RegisterCount) ];
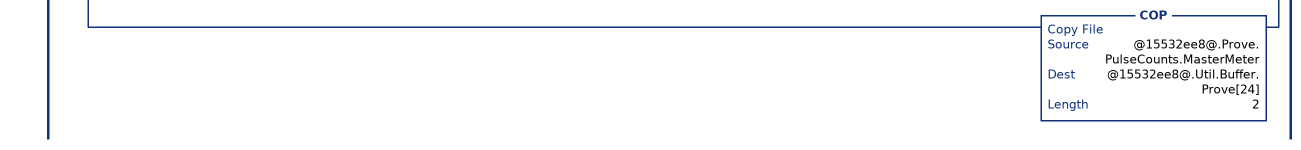
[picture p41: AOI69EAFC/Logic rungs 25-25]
   // The reason to check NEQ outputbuffer[0] 5000 is to guarantee the routine will be updated one time only, so the signals can be cleared correctly once the input block is received
   25: XIC(@15532ee8@.Prove.ProveEnabled)[NEQ(@15532ee8@.Util.Buffer.Output[0],5000) ,OTL(@15532ee8@.Util.Block.NonInterruptPending.Prover) ]EQU(@15532ee8@.Util.CycleCounter,5000)[MOV(0,@9564c3a6@) ,XIC(@15532ee8@.Prove.Process.Sequencing.Phase.NotSelected) [OTU(@9564c3a6@.0) ,OTU(@9564c3a6@.1) ,OTU(@9564c3a6@.2) ] ,XIC(@15532ee8@.Prove.Process.Sequencing.Phase.Active) [OTL(@9564c3a6@.0) ,OTU(@9564c3a6@.1) ,OTU(@9564c3a6@.2) ] ,XIC(@15532ee8@.Prove.Process.Sequencing.Phase.CountingPast1stSwitch) [OTU(@9564c3a6@.0) ,OTL(@9564c3a6@.1) ,OTU(@9564c3a6@.2) ] ,XIC(@15532ee8@.Prove.Process.Sequencing.Phase.Past2ndSwitchFwdLeg) [OTL(@9564c3a6@.0) ,OTL(@9564c3a6@.1) ,OTU(@9564c3a6@.2) ] ,XIC(@15532ee8@.Prove.Process.Sequencing.Phase.Past1stSwithRetLeg) [OTU(@9564c3a6@.0) ,OTU(@9564c3a6@.1) ,OTL(@9564c3a6@.2) ] ,XIC(@15532ee8@.Prove.Process.Sequencing.Phase.RunComplete) [OTL(@9564c3a6@.0) ,OTU(@9564c3a6@.1) ,OTL(@9564c3a6@.2) ] ,NEQ(@9564c3a6@,1) NEQ(@9564c3a6@,2) NEQ(@9564c3a6@,3) NEQ(@9564c3a6@,4) NEQ(@9564c3a6@,5) [OTL(@15532ee8@.Prove.Process.Sequencing.Phase.NotSelected) ,OTU(@15532ee8@.Prove.Process.Sequencing.Phase.Active) ,OTU(@15532ee8@.Prove.Process.Sequencing.Phase.CountingPast1stSwitch) ,OTU(@15532ee8@.Prove.Process.Sequencing.Phase.Past2ndSwitchFwdLeg) ,OTU(@15532ee8@.Prove.Process.Sequencing.Phase.Past1stSwithRetLeg) ,OTU(@15532ee8@.Prove.Process.Sequencing.Phase.RunComplete) ,MOV(0,@9564c3a6@) ] ,XIC(@15532ee8@.Prove.Process.Sequencing.BallPositionReady) OTL(@9564c3a6@.8) ,XIC(@15532ee8@.Prove.Process.Sequencing.BallPositionSealed) OTL(@9564c3a6@.9) ,XIC(@15532ee8@.Prove.Process.Sequencing.BallPositionReadyBwdLeg) OTL(@9564c3a6@.10) ,XIC(@15532ee8@.Prove.Process.Sequencing.BallPositionSealedBwdLeg) OTL(@9564c3a6@.11) ,MOV(16#7C00,@15532ee8@.Util.Buffer.Prove[0]) ,MOV(@9564c3a6@,@15532ee8@.Util.Buffer.Prove[1]) ,COP(@15532ee8@.Prove.Process.Temperature,@15532ee8@.Util.Buffer.Prove[4],2) ,COP(@15532ee8@.Prove.Process.OutletTemperature,@15532ee8@.Util.Buffer.Prove[6],2) ,COP(@15532ee8@.Prove.Process.SwitchBarTemperature,@15532ee8@.Util.Buffer.Prove[8],2) ,COP(@15532ee8@.Prove.Process.Pressure,@15532ee8@.Util.Buffer.Prove[10],2) ,COP(@15532ee8@.Prove.Process.OutletPressure,@15532ee8@.Util.Buffer.Prove[12],2) ,COP(@15532ee8@.Prove.Process.ProverDensity,@15532ee8@.Util.Buffer.Prove[14],2) ,MOV(0,@f8aaafbf@) ,XIC(@15532ee8@.Prove.Signals.EnableProve) OTL(@f8aaafbf@.1) ,XIC(@15532ee8@.Prove.Signals.AcceptProve) OTL(@f8aaafbf@.2) ,XIC(@15532ee8@.Prove.Signals.RejectProve) OTL(@f8aaafbf@.3) ,XIC(@15532ee8@.Prove.Signals.RunStart) OTL(@f8aaafbf@.4) ,XIC(@15532ee8@.Prove.Signals.RunComplete) OTL(@f8aaafbf@.5) ,XIC(@15532ee8@.Prove.Signals.RunCancel) OTL(@f8aaafbf@.6) ,XIC(@15532ee8@.Prove.Signals.RunDelete) OTL(@f8aaafbf@.7) ,XIC(@15532ee8@.Prove.Signals.PassComplete) OTL(@f8aaafbf@.9) ,XIC(@15532ee8@.Prove.Signals.PauseProve) OTL(@f8aaafbf@.12) ,XIC(@15532ee8@.Prove.Signals.AbortProve) OTL(@f8aaafbf@.14) ,MOV(@f8aaafbf@,@15532ee8@.Util.Buffer.Prove[16]) ,[MOV(0,@8cad0451@) ,XIC(@15532ee8@.Prove.Config.Enable.AutoAcceptProve) OTL(@8cad0451@.0) ,XIC(@15532ee8@.Prove.Config.Enable.AutoContinueProve) OTL(@8cad0451@.1) ,XIC(@15532ee8@.Prove.Config.Accept.ApplyMFChangeAllStreams) OTL(@8cad0451@.13) ,XIC(@15532ee8@.Prove.Config.Accept.ApplyMFChangeCurve) OTL(@8cad0451@.14) ,XIC(@15532ee8@.Prove.Config.Accept.ApplyNewMF) OTL(@8cad0451@.15) ,MOV(@8cad0451@,@15532ee8@.Util.Buffer.Prove[17]) ,MOV(@15532ee8@.Prove.Config.Enable.MeterNumber,@15532ee8@.Util.Buffer.Prove[18]) ,MOV(@15532ee8@.Prove.Config.Accept.RequestedInterpolationPoint,@15532ee8@.Util.Buffer.Prove[21]) ] ,[COP(@15532ee8@.Prove.PulseCounts.Meter,@15532ee8@.Util.Buffer.Prove[22],2) ,COP(@15532ee8@.Prove.PulseCounts.MasterMeter,@15532ee8@.Util.Buffer.Prove[24],2) ] ];
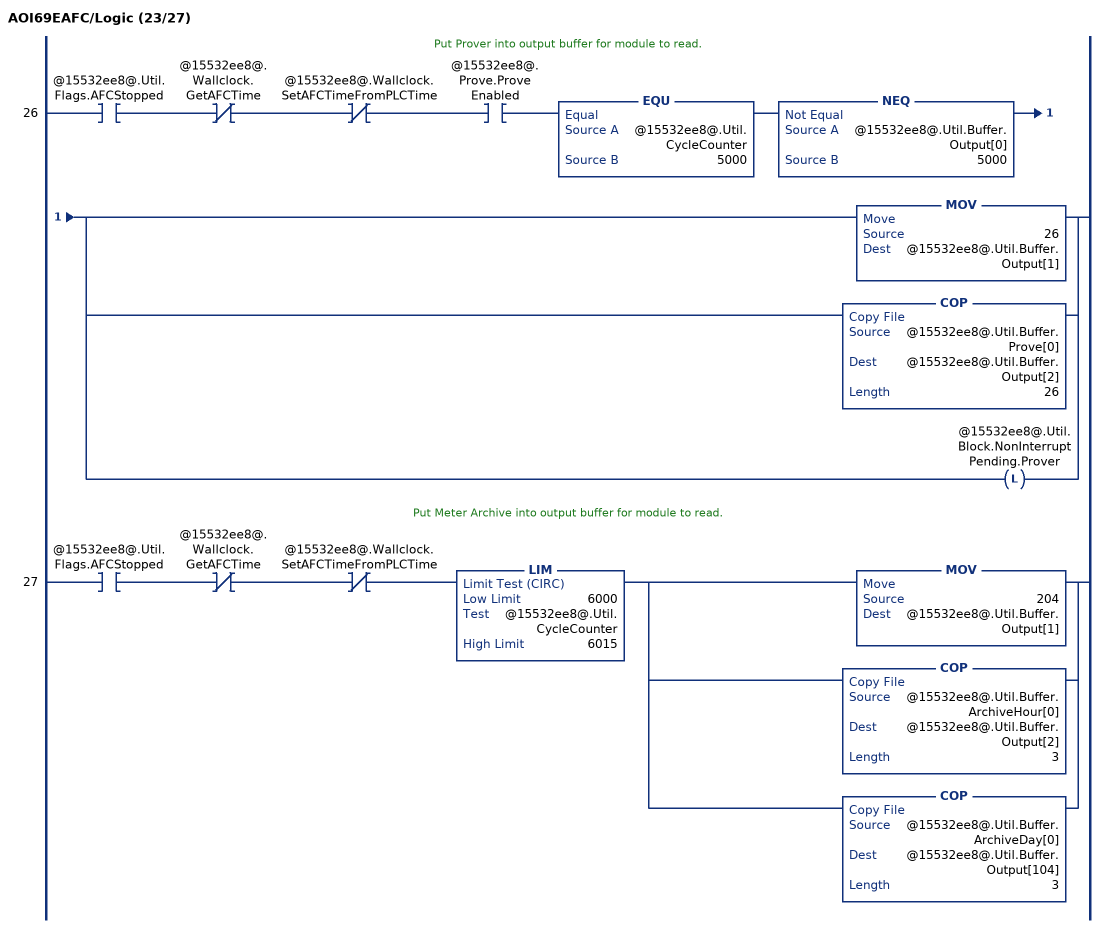
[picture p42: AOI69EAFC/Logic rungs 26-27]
   // Put Prover into output buffer for module to read.
   26: XIC(@15532ee8@.Util.Flags.AFCStopped)XIO(@15532ee8@.Wallclock.GetAFCTime)XIO(@15532ee8@.Wallclock.SetAFCTimeFromPLCTime)XIC(@15532ee8@.Prove.ProveEnabled)EQU(@15532ee8@.Util.CycleCounter,5000)NEQ(@15532ee8@.Util.Buffer.Output[0],5000)[MOV(26,@15532ee8@.Util.Buffer.Output[1]) ,COP(@15532ee8@.Util.Buffer.Prove[0],@15532ee8@.Util.Buffer.Output[2],26) ,OTL(@15532ee8@.Util.Block.NonInterruptPending.Prover) ];
   // Put Meter Archive into output buffer for module to read.
   27: XIC(@15532ee8@.Util.Flags.AFCStopped)XIO(@15532ee8@.Wallclock.GetAFCTime)XIO(@15532ee8@.Wallclock.SetAFCTimeFromPLCTime)LIM(6000,@15532ee8@.Util.CycleCounter,6015)[MOV(204,@15532ee8@.Util.Buffer.Output[1]) ,COP(@15532ee8@.Util.Buffer.ArchiveHour[0],@15532ee8@.Util.Buffer.Output[2],3) ,COP(@15532ee8@.Util.Buffer.ArchiveDay[0],@15532ee8@.Util.Buffer.Output[104],3) ];
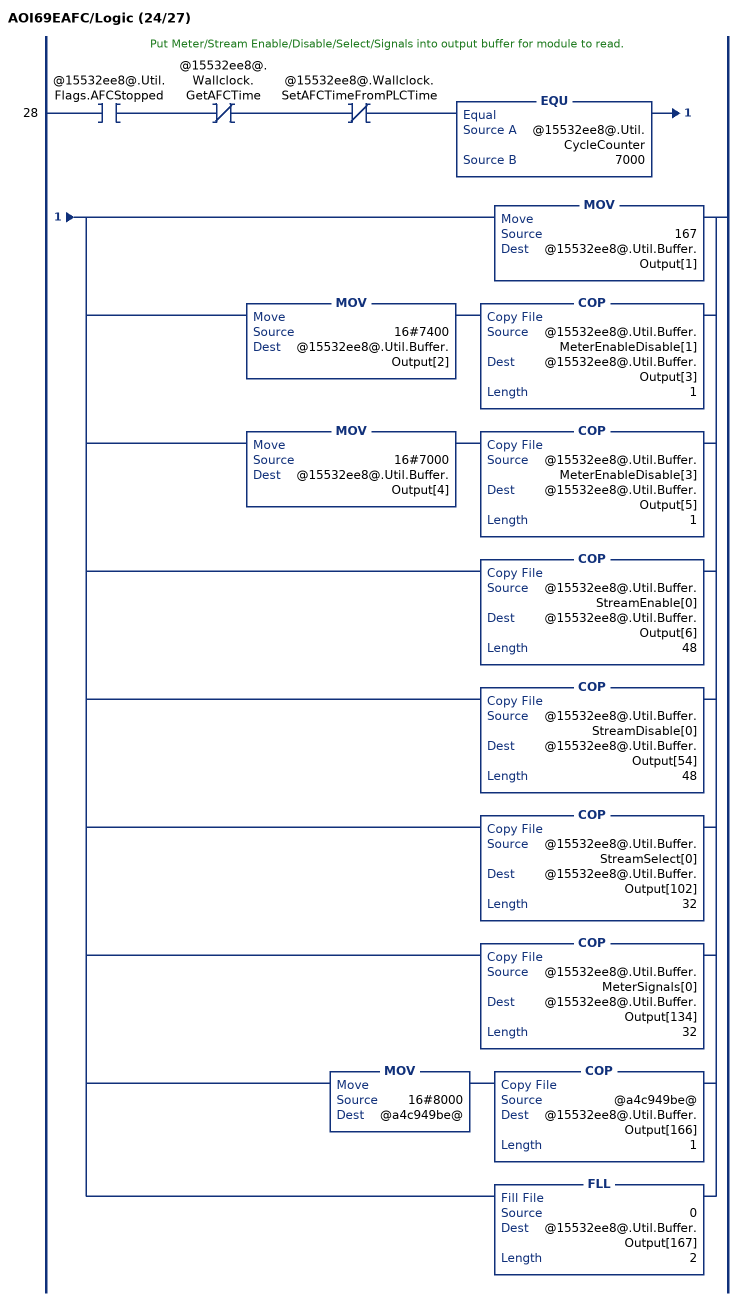
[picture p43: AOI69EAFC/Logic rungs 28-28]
   // Put Meter/Stream Enable/Disable/Select/Signals into output buffer for module to read.
   28: XIC(@15532ee8@.Util.Flags.AFCStopped)XIO(@15532ee8@.Wallclock.GetAFCTime)XIO(@15532ee8@.Wallclock.SetAFCTimeFromPLCTime)EQU(@15532ee8@.Util.CycleCounter,7000)[MOV(167,@15532ee8@.Util.Buffer.Output[1]) ,MOV(16#7400,@15532ee8@.Util.Buffer.Output[2]) COP(@15532ee8@.Util.Buffer.MeterEnableDisable[1],@15532ee8@.Util.Buffer.Output[3],1) ,MOV(16#7000,@15532ee8@.Util.Buffer.Output[4]) COP(@15532ee8@.Util.Buffer.MeterEnableDisable[3],@15532ee8@.Util.Buffer.Output[5],1) ,COP(@15532ee8@.Util.Buffer.StreamEnable[0],@15532ee8@.Util.Buffer.Output[6],48) ,COP(@15532ee8@.Util.Buffer.StreamDisable[0],@15532ee8@.Util.Buffer.Output[54],48) ,COP(@15532ee8@.Util.Buffer.StreamSelect[0],@15532ee8@.Util.Buffer.Output[102],32) ,COP(@15532ee8@.Util.Buffer.MeterSignals[0],@15532ee8@.Util.Buffer.Output[134],32) ,[MOV(16#8000,@a4c949be@) COP(@a4c949be@,@15532ee8@.Util.Buffer.Output[166],1) ,FLL(0,@15532ee8@.Util.Buffer.Output[167],2) ] ];
